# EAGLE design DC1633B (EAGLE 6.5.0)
PROGRAMMABLE HEX VOLTAGE SUPERVISOR WITH EEPROM

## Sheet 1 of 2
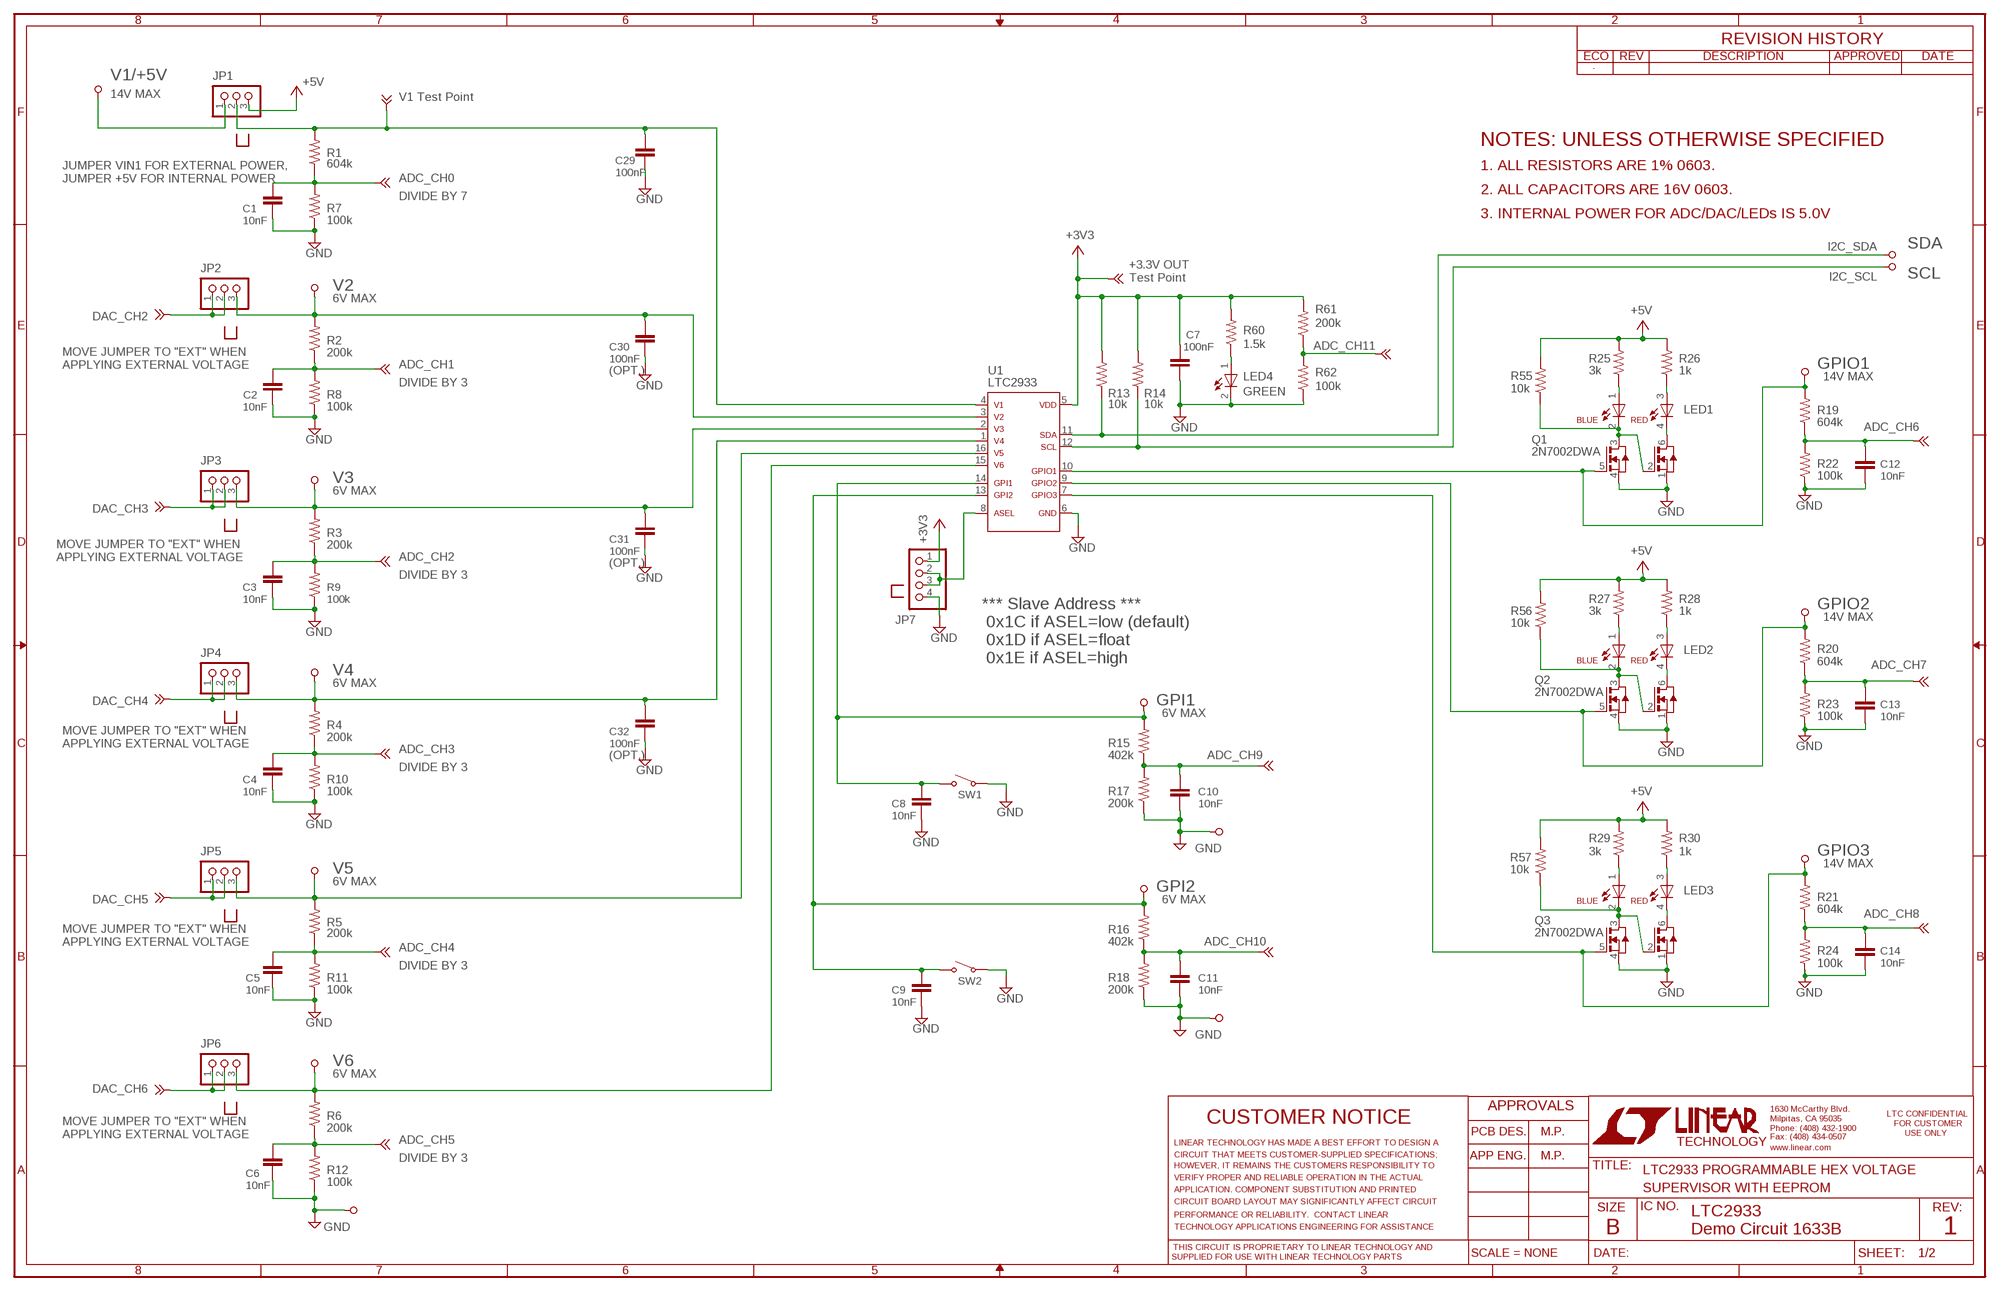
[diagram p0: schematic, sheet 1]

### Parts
C1  10nF  CC0603_BOX  [C0603_BOX]
C2  10nF  CC0603_BOX  [C0603_BOX]
C3  10nF  CC0603_BOX  [C0603_BOX]
C4  10nF  CC0603_BOX  [C0603_BOX]
C5  10nF  CC0603_BOX  [C0603_BOX]
C6  10nF  CC0603_BOX  [C0603_BOX]
C7  100nF  CC0603_BOX  [C0603_BOX]
C8  10nF  CC0603_BOX  [C0603_BOX]
C9  10nF  CC0603_BOX  [C0603_BOX]
C10  10nF  CC0603_BOX  [C0603_BOX]
C11  10nF  CC0603_BOX  [C0603_BOX]
C12  10nF  CC0603_BOX  [C0603_BOX]
C13  10nF  CC0603_BOX  [C0603_BOX]
C14  10nF  CC0603_BOX  [C0603_BOX]
C29  100nF  CC0603_BOX  [C0603_BOX]
C30  100nF  CC0603_BOX  [C0603_BOX]
C31  100nF  CC0603_BOX  [C0603_BOX]
C32  100nF  CC0603_BOX  [C0603_BOX]
JP1  NRPN031PAEN-RC  PINHD-1X3  [1X03]
JP2  NRPN031PAEN-RC  PINHD-1X3  [1X03]
JP3  NRPN031PAEN-RC  PINHD-1X3  [1X03]
JP4  NRPN031PAEN-RC  PINHD-1X3  [1X03]
JP5  NRPN031PAEN-RC  PINHD-1X3  [1X03]
JP6  NRPN031PAEN-RC  PINHD-1X3  [1X03]
JP7  NRPN041PAEN-RC  PINHD-1X4-2MM  [1X04-2MM]
LED1  LED-DUAL-COLOR_1.6X0.8MM  [LED-DUAL_1.6X0.8MM]
LED2  LED-DUAL-COLOR_1.6X0.8MM  [LED-DUAL_1.6X0.8MM]
LED3  LED-DUAL-COLOR_1.6X0.8MM  [LED-DUAL_1.6X0.8MM]
LED4  LED-0603  [CHIPLED_0603]
Q1  2N7002DWA  [SOT-363]
Q2  2N7002DWA  [SOT-363]
Q3  2N7002DWA  [SOT-363]
R1  604k  RR0603_BOX  [R0603_BOX]
R2  200k  RR0603_BOX  [R0603_BOX]
R3  200k  RR0603_BOX  [R0603_BOX]
R4  200k  RR0603_BOX  [R0603_BOX]
R5  200k  RR0603_BOX  [R0603_BOX]
R6  200k  RR0603_BOX  [R0603_BOX]
R7  100k  RR0603_BOX  [R0603_BOX]
R8  100k  RR0603_BOX  [R0603_BOX]
R9  100k  RR0603_BOX  [R0603_BOX]
R10  100k  RR0603_BOX  [R0603_BOX]
R11  100k  RR0603_BOX  [R0603_BOX]
R12  100k  RR0603_BOX  [R0603_BOX]
R13  10k  RR0603_BOX  [R0603_BOX]
R14  10k  RR0603_BOX  [R0603_BOX]
R15  402k  RR0603_BOX  [R0603_BOX]
R16  402k  RR0603_BOX  [R0603_BOX]
R17  200k  RR0603_BOX  [R0603_BOX]
R18  200k  RR0603_BOX  [R0603_BOX]
R19  604k  RR0603_BOX  [R0603_BOX]
R20  604k  RR0603_BOX  [R0603_BOX]
R21  604k  RR0603_BOX  [R0603_BOX]
R22  100k  RR0603_BOX  [R0603_BOX]
R23  100k  RR0603_BOX  [R0603_BOX]
R24  100k  RR0603_BOX  [R0603_BOX]
R25  3k  RR0603_BOX  [R0603_BOX]
R26  1k  RR0603_BOX  [R0603_BOX]
R27  3k  RR0603_BOX  [R0603_BOX]
R28  1k  RR0603_BOX  [R0603_BOX]
R29  3k  RR0603_BOX  [R0603_BOX]
R30  1k  RR0603_BOX  [R0603_BOX]
R55  10k  RR0603_BOX  [R0603_BOX]
R56  10k  RR0603_BOX  [R0603_BOX]
R57  10k  RR0603_BOX  [R0603_BOX]
R60  1.5k  RR0603_BOX  [R0603_BOX]
R61  200k  RR0603_BOX  [R0603_BOX]
R62  100k  RR0603_BOX  [R0603_BOX]
SW1  SWITCH_PTS635  [SWITCH_PTS635]
SW2  SWITCH_PTS635  [SWITCH_PTS635]
TP1  TESTPOINT_BIG  [TP1]
TP2  TESTPOINT_BIG  [TP1]
TP3  TESTPOINT_BIG  [TP1]
TP4  TESTPOINT_BIG  [TP1]
TP5  TESTPOINT_BIG  [TP1]
TP6  TESTPOINT_BIG  [TP1]
TP7  TESTPOINT_BIG  [TP1]
TP8  TESTPOINT_BIG  [TP1]
TP9  TESTPOINT_BIG  [TP1]
TP10  TESTPOINT_BIG  [TP1]
TP11  TESTPOINT_BIG  [TP1]
TP12  TESTPOINT_BIG  [TP1]
TP13  TESTPOINT_BIG  [TP1]
TP14  TESTPOINT_BIG  [TP1]
TP15  TESTPOINT_BIG  [TP1]
TP16  TESTPOINT_BIG  [TP1]
TP20  TESPOINT_SMDVIA  [VIA]
TP21  TESPOINT_SMDVIA  [VIA]
U1  LTC2933  [SSOP16]

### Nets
+3V3: C7.1 JP7.1 R13.2 R14.2 R60.2 R61.2 TP20.1 U1.5
+5V: JP1.3 R25.2 R26.2 R27.2 R28.2 R29.2 R30.2 R55.2 R56.2 R57.2 ; also sheet 2
ADC_CH0: C1.1 R1.1 R7.2 ; also sheet 2
ADC_CH1: C2.1 R2.1 R8.2 ; also sheet 2
ADC_CH2: C3.1 R3.1 R9.2 ; also sheet 2
ADC_CH3: C4.1 R4.1 R10.2 ; also sheet 2
ADC_CH4: C5.1 R5.1 R11.2 ; also sheet 2
ADC_CH5: C6.1 R6.1 R12.2 ; also sheet 2
ADC_CH6: C12.1 R19.1 R22.2 ; also sheet 2
ADC_CH7: C13.1 R20.1 R23.2 ; also sheet 2
ADC_CH8: C14.1 R21.1 R24.2 ; also sheet 2
ADC_CH9: C10.1 R15.1 R17.2 ; also sheet 2
ADC_CH10: C11.1 R16.1 R18.2 ; also sheet 2
ADC_CH11: R61.1 R62.2 ; also sheet 2
DAC_CH2: JP2.1 JP2.2 ; also sheet 2
DAC_CH3: JP3.1 JP3.2 ; also sheet 2
DAC_CH4: JP4.1 JP4.2 ; also sheet 2
DAC_CH5: JP5.1 JP5.2 ; also sheet 2
DAC_CH6: JP6.1 JP6.2 ; also sheet 2
GND: C1.2 C2.2 C3.2 C4.2 C5.2 C6.2 C7.2 C8.2 C9.2 C10.2 C11.2 C12.2 C13.2 C14.2 C29.2 C30.2 C31.2 C32.2 JP7.4 LED4.N(C) Q1.1(S2) Q1.4(S1) Q2.1(S2) Q2.4(S1) Q3.1(S2) Q3.4(S1) R7.1 R8.1 R9.1 R10.1 R11.1 R12.1 R17.1 R18.1 R22.1 R23.1 R24.1 R62.1 SW1.SW2 SW2.SW2 TP14.TP TP15.TP TP16.TP U1.6 ; also sheet 2
I2C_SCL: R14.1 TP13.TP U1.12 ; also sheet 2
I2C_SDA: R13.1 TP12.TP U1.11 ; also sheet 2
N$15: LED4.P(A) R60.1
N$17: JP1.1 TP1.TP
N$20: C29.1 JP1.2 R1.2 TP21.1 U1.4
N$26: JP7.2 JP7.3 U1.8
N$32: Q2.5(G1) R20.2 TP8.TP U1.9
N$34: LED1.4(C4) Q1.6(D2)
N$36: LED2.2(C2) Q2.2(G2) Q2.3(D1) R56.1
N$37: LED3.2(C2) Q3.2(G2) Q3.3(D1) R57.1
N$38: LED1.2(C2) Q1.2(G2) Q1.3(D1) R55.1
N$40: Q3.5(G1) R21.2 TP9.TP U1.7
N$41: Q1.5(G1) R19.2 TP7.TP U1.10
N$44: LED3.4(C4) Q3.6(D2)
N$45: LED3.1(A1) R29.1
N$47: LED3.3(A3) R30.1
N$49: LED2.4(C4) Q2.6(D2)
N$50: LED2.1(A1) R27.1
N$51: LED2.3(A3) R28.1
N$54: LED1.1(A1) R25.1
N$55: LED1.3(A3) R26.1
N$77: C8.1 R15.2 SW1.SW1 TP10.TP U1.14
N$78: C9.1 R16.2 SW2.SW1 TP11.TP U1.13
VIN2: C30.1 JP2.3 R2.2 TP2.TP U1.3
VIN3: C31.1 JP3.3 R3.2 TP3.TP U1.2
VIN4: C32.1 JP4.3 R4.2 TP4.TP U1.1
VIN5: JP5.3 R5.2 TP5.TP U1.16
VIN6: JP6.3 R6.2 TP6.TP U1.15

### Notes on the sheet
- V1/+5V
- 14V MAX | V1 Test Point
- NOTES: UNLESS OTHERWISE SPECIFIED
- 1. ALL RESISTORS ARE 1% 0603.
- JUMPER VIN1 FOR EXTERNAL POWER,
  JUMPER +5V FOR INTERNAL POWER
- 2. ALL CAPACITORS ARE 16V 0603.
- DIVIDE BY 7
- 3. INTERNAL POWER FOR ADC/DAC/LEDs IS 5.0V
- SDA
- SCL
- +3.3V OUT
  Test Point
- V2
- 6V MAX
- MOVE JUMPER TO "EXT" WHEN
  APPLYING EXTERNAL VOLTAGE
- GPIO1
- (OPT.)
- 14V MAX
- DIVIDE BY 3
- GREEN
- V3
- 6V MAX
- MOVE JUMPER TO "EXT" WHEN
  APPLYING EXTERNAL VOLTAGE
- (OPT.)
- DIVIDE BY 3
- GPIO2
- 14V MAX
- *** Slave Address ***
   0x1C if ASEL=low (default)
   0x1D if ASEL=float
   0x1E if ASEL=high
- V4
- 6V MAX
- GPI1
- 6V MAX
- MOVE JUMPER TO "EXT" WHEN
  APPLYING EXTERNAL VOLTAGE
- (OPT.)
- DIVIDE BY 3
- GPIO3
- 14V MAX
- V5
- 6V MAX
- GPI2
- 6V MAX
- MOVE JUMPER TO "EXT" WHEN
  APPLYING EXTERNAL VOLTAGE
- DIVIDE BY 3
- V6
- 6V MAX
- M.P.
- MOVE JUMPER TO "EXT" WHEN
  APPLYING EXTERNAL VOLTAGE
- DIVIDE BY 3 | M.P.
- LTC2933 PROGRAMMABLE HEX VOLTAGE
- SUPERVISOR WITH EEPROM
- LTC2933
- Demo Circuit 1633B | 1

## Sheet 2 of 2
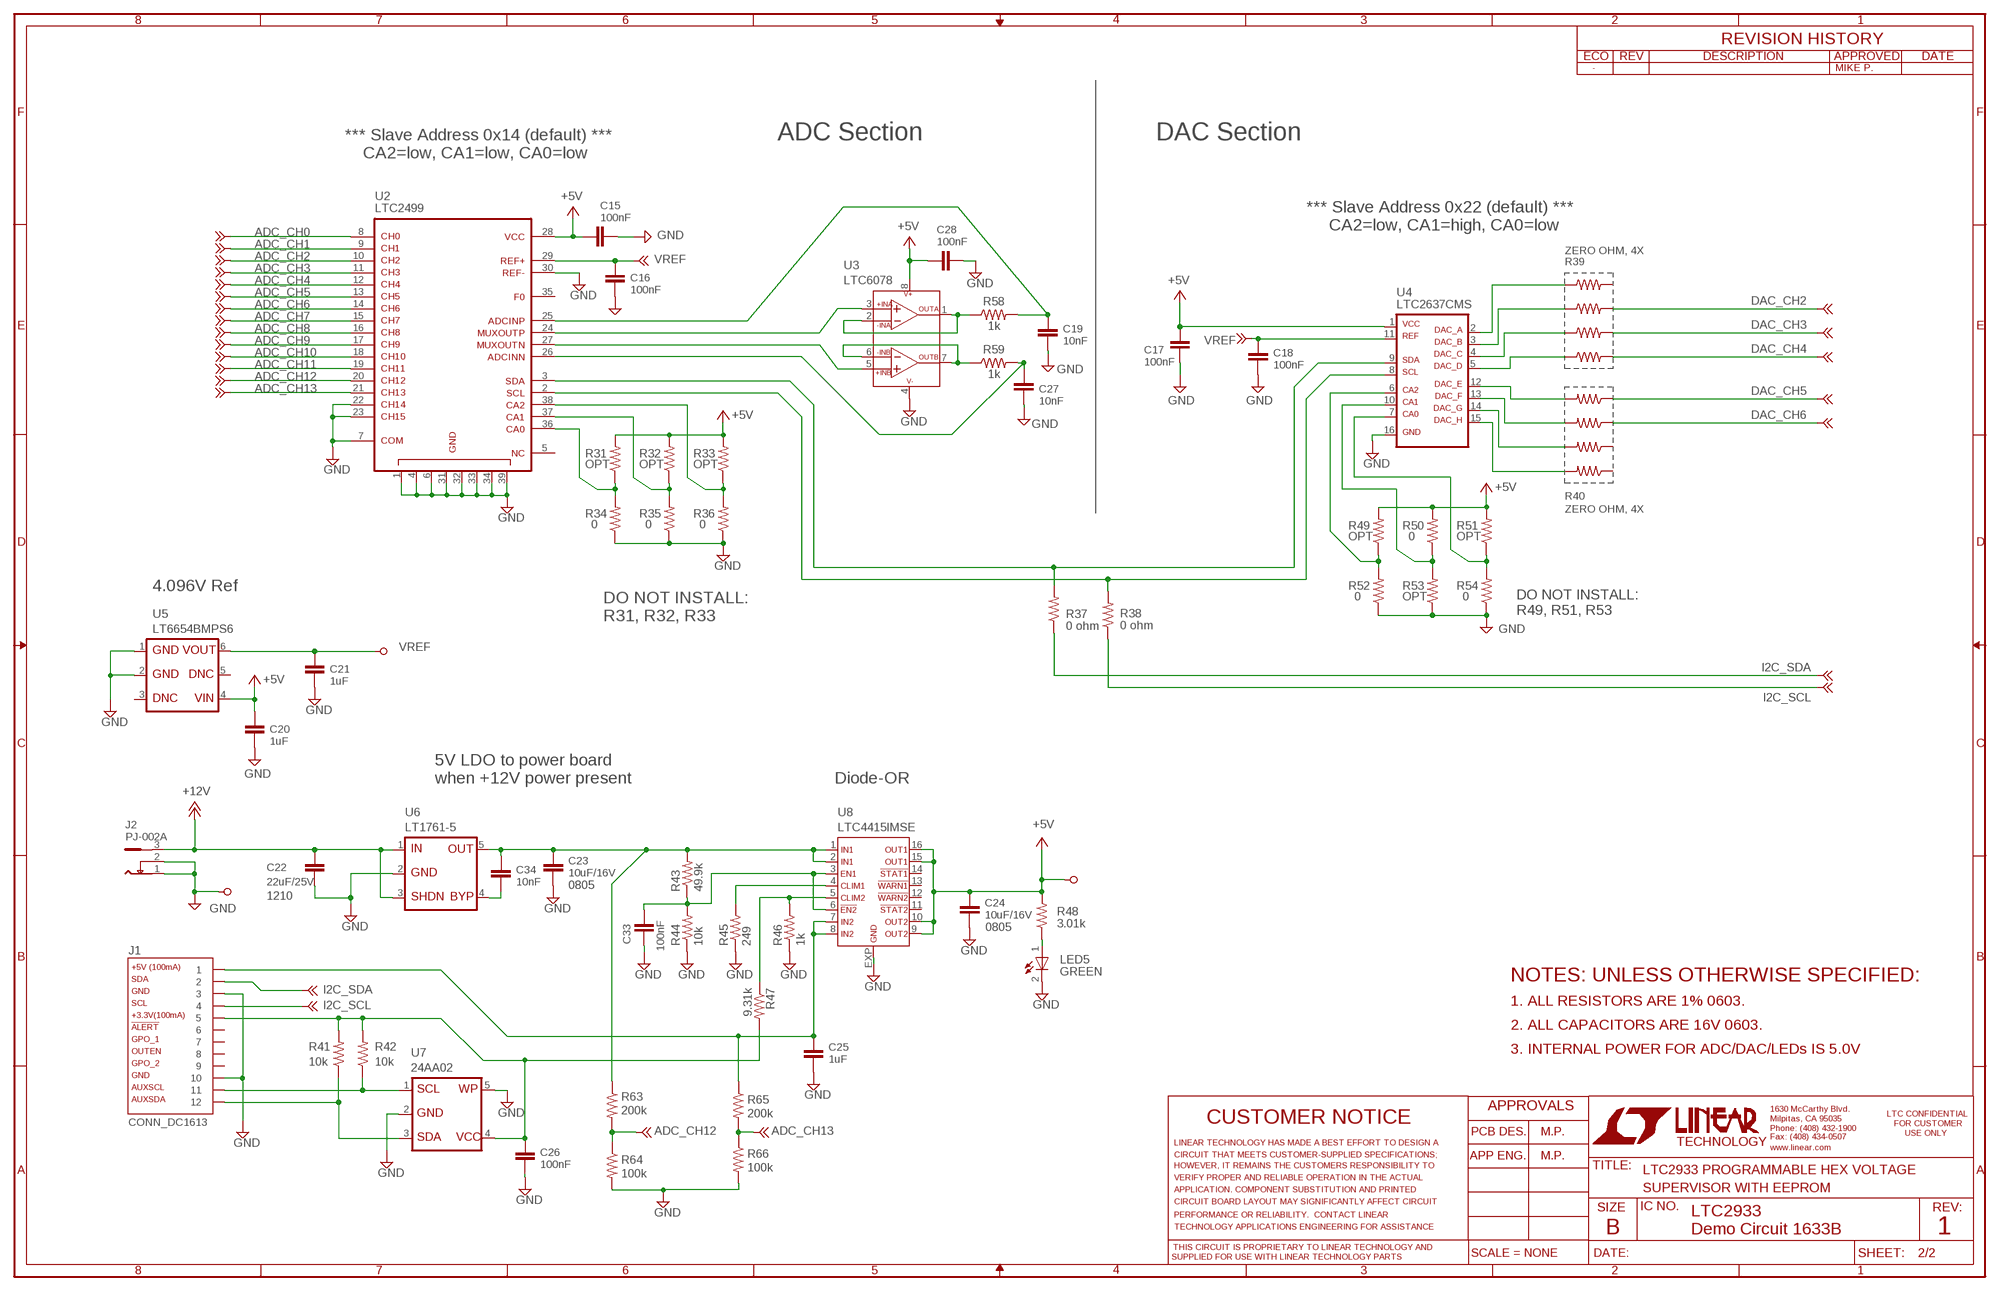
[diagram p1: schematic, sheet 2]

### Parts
C15  100nF  CC0603_BOX  [C0603_BOX]
C16  100nF  CC0603_BOX  [C0603_BOX]
C17  100nF  CC0603_BOX  [C0603_BOX]
C18  100nF  CC0603_BOX  [C0603_BOX]
C19  10nF  CC0603_BOX  [C0603_BOX]
C20  1uF  CC0603_BOX  [C0603_BOX]
C21  1uF  CC0603_BOX  [C0603_BOX]
C22  22uF/25V  CC1210_BOX  [C1210_BOX]
C23  10uF/16V  CC0805_BOX  [C0805_BOX]
C24  10uF/16V  CC0805_BOX  [C0805_BOX]
C25  1uF  CC0603_BOX  [C0603_BOX]
C26  100nF  CC0603_BOX  [C0603_BOX]
C27  10nF  CC0603_BOX  [C0603_BOX]
C28  100nF  CC0603_BOX  [C0603_BOX]
C33  100nF  CC0603_BOX  [C0603_BOX]
C34  10nF  CC0603_BOX  [C0603_BOX]
J1  CONN_DC1613  [CONN_DC1613]
J2  PJ-002A  [PJ-002A]
LED5  LED-0603  [CHIPLED_0603]
R31  OPT  RR0603_BOX  [R0603_BOX]
R32  OPT  RR0603_BOX  [R0603_BOX]
R33  OPT  RR0603_BOX  [R0603_BOX]
R34  0  RR0603_BOX  [R0603_BOX]
R35  0  RR0603_BOX  [R0603_BOX]
R36  0  RR0603_BOX  [R0603_BOX]
R37  0 ohm  RR0603_BOX  [R0603_BOX]
R38  0 ohm  RR0603_BOX  [R0603_BOX]
R39  R_ARRAY_4X_CRA06S  [R_VISHAY_CRA06S]
R40  R_ARRAY_4X_CRA06S  [R_VISHAY_CRA06S]
R41  10k  RR0603_BOX  [R0603_BOX]
R42  10k  RR0603_BOX  [R0603_BOX]
R43  49.9k  RR0603_BOX  [R0603_BOX]
R44  10k  RR0603_BOX  [R0603_BOX]
R45  249  RR0603_BOX  [R0603_BOX]
R46  1k  RR0603_BOX  [R0603_BOX]
R47  9.31k  RR0603_BOX  [R0603_BOX]
R48  3.01k  RR0603_BOX  [R0603_BOX]
R49  OPT  RR0603_BOX  [R0603_BOX]
R50  0  RR0603_BOX  [R0603_BOX]
R51  OPT  RR0603_BOX  [R0603_BOX]
R52  0  RR0603_BOX  [R0603_BOX]
R53  OPT  RR0603_BOX  [R0603_BOX]
R54  0  RR0603_BOX  [R0603_BOX]
R58  1k  RR0603_BOX  [R0603_BOX]
R59  1k  RR0603_BOX  [R0603_BOX]
R63  200k  RR0603_BOX  [R0603_BOX]
R64  100k  RR0603_BOX  [R0603_BOX]
R65  200k  RR0603_BOX  [R0603_BOX]
R66  100k  RR0603_BOX  [R0603_BOX]
TP17  TESTPOINT_BIG  [TP1]
TP18  TESTPOINT_BIG  [TP1]
TP19  TURRET_SMALL_2308TP  [TURRET_SMALL_2308]
TP24  TESPOINT_SMDVIA  [VIA]
TP25  TESPOINT_SMDVIA  [VIA]
TP26  TESPOINT_SMDVIA  [VIA]
TP27  TESPOINT_SMDVIA  [VIA]
TP28  TESPOINT_SMDVIA  [VIA]
TP29  TESPOINT_SMDVIA  [VIA]
TP33  TESPOINT_SMDVIA  [VIA]
TP34  TESPOINT_SMDVIA  [VIA]
U2  LTC2499  [QFN38_5X7]
U3  LTC6078  [MSOP8]
U4  LTC2637CMS  [MSOP16]
U5  LT6654BMPS6  [SOT-23-6]
U6  LT1761-5  [SOT-23-5]
U7  24AA02  [SOT-23-5]
U8  LTC4415IMSE  [MSOP16_EXP]

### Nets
+5V: C15.1 C17.1 C20.1 C24.1 C28.1 R31.2 R32.2 R33.2 R48.2 R49.2 R50.2 R51.2 TP18.TP U2.28 U3.8 U4.1 U5.4 U8.9 U8.10 U8.15 U8.16 ; also sheet 1
+12V: C22.1 J2.3 U6.1 U6.3
ADC_CH0: TP24.1 U2.8 ; also sheet 1
ADC_CH1: TP25.1 U2.9 ; also sheet 1
ADC_CH2: TP26.1 U2.10 ; also sheet 1
ADC_CH3: TP27.1 U2.11 ; also sheet 1
ADC_CH4: TP28.1 U2.12 ; also sheet 1
ADC_CH5: TP29.1 U2.13 ; also sheet 1
ADC_CH6: U2.14 ; also sheet 1
ADC_CH7: U2.15 ; also sheet 1
ADC_CH8: U2.16 ; also sheet 1
ADC_CH9: TP33.1 U2.17 ; also sheet 1
ADC_CH10: TP34.1 U2.18 ; also sheet 1
ADC_CH11: U2.19 ; also sheet 1
ADC_CH12: R63.2 R64.1 U2.20
ADC_CH13: R65.2 R66.1 U2.21
DAC_CH2: R39.R2_2 ; also sheet 1
DAC_CH3: R39.R3_2 ; also sheet 1
DAC_CH4: R39.R4_2 ; also sheet 1
DAC_CH5: R40.R4_1 ; also sheet 1
DAC_CH6: R40.R3_1 ; also sheet 1
GND: C15.2 C16.2 C17.2 C18.2 C19.2 C20.2 C21.2 C22.2 C23.2 C24.2 C25.2 C26.2 C27.2 C28.2 C33.2 J1.3 J1.10 J2.1 J2.2 LED5.N(C) R34.1 R35.1 R36.1 R44.1 R45.1 R46.1 R52.1 R53.1 R54.1 R64.2 R66.2 TP17.TP U2.1(GND1) U2.4(GND4) U2.6(GND6) U2.7 U2.22 U2.23 U2.30 U2.31(GND31) U2.32(GND32) U2.33(GND33) U2.34(GND34) U2.39(GND39) U3.4 U4.16 U5.1 U5.2 U6.2 U7.2 U7.5 U8.EXP ; also sheet 1
I2C_SCL: J1.4 R38.1 ; also sheet 1
I2C_SDA: J1.2 R37.1 ; also sheet 1
N$1: R40.R4_2 U4.12
N$2: R50.1 R53.2 U4.10
N$3: R40.R3_2 U4.13
N$4: R51.1 R54.2 U4.7
N$5: R40.R2_2 U4.14
N$6: R49.1 R52.2 U4.6
N$7: R40.R1_2 U4.15
N$9: R39.R4_1 U4.5
N$10: LED5.P(A) R48.1
N$11: R39.R3_1 U4.4
N$12: C23.1 C34.1 R43.2 R63.1 U6.5 U8.1 U8.2
N$13: R39.R2_1 U4.3
N$14: C33.1 R43.1 R44.2 U8.3 U8.6
N$16: R58.1 U3.1 U3.2
N$18: R39.R1_1 U4.2
N$19: R38.2 U2.2 U4.8
N$21: R45.2 U8.4
N$22: R46.2 R47.1 U8.5
N$23: C34.2 U6.4
N$24: J1.11 R42.1 U7.1
N$25: J1.12 R41.1 U7.3
N$27: R32.1 R35.2 U2.37
N$28: R31.1 R34.2 U2.36
N$29: R37.2 U2.3 U4.9
N$30: R33.1 R36.2 U2.38
N$31: U2.24 U3.3
N$33: U2.27 U3.5
N$39: R59.1 U3.6 U3.7
N$43: C26.1 J1.5 R41.2 R42.2 R47.2 U7.4
N$46: C27.1 R59.2 U2.26
N$48: C19.1 R58.2 U2.25
USB_5V: C25.1 J1.1 R65.1 U8.7 U8.8
VREF: C16.1 C18.1 C21.1 TP19.TP1 U2.29 U4.11 U5.6
Unconnected: J1.6 J1.7 J1.8 J1.9 R39.R1_2 R40.R1_1 R40.R2_1 U2.5 U2.35 U5.3 U5.5 U8.11 U8.12 U8.13 U8.14

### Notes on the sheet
- MIKE P.
- ADC Section | DAC Section
- *** Slave Address 0x14 (default) ***
      CA2=low, CA1=low, CA0=low
- *** Slave Address 0x22 (default) ***
       CA2=low, CA1=high, CA0=low
- ZERO OHM, 4X
- ZERO OHM, 4X
- 4.096V Ref
- DO NOT INSTALL:
  R49, R51, R53
- DO NOT INSTALL:
  R31, R32, R33
- 5V LDO to power board
  when +12V power present
- Diode-OR
- 0805
- 1210
- 0805
- GREEN
- NOTES: UNLESS OTHERWISE SPECIFIED:
- 1. ALL RESISTORS ARE 1% 0603.
- 2. ALL CAPACITORS ARE 16V 0603.
- 3. INTERNAL POWER FOR ADC/DAC/LEDs IS 5.0V
- M.P.
- M.P.
- LTC2933 PROGRAMMABLE HEX VOLTAGE
- SUPERVISOR WITH EEPROM
- LTC2933
- Demo Circuit 1633B | 1

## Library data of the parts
C1-C34 = kalin:C: CAPACITOR, European symbol
J1 = kalin:CONN_DC1613: Connector for LT DC1613 USB Dongle
J2 = kalin:PJ-002A: Power Jack from CUI Inc. PJ-002A
JP1-JP6 = pinhead:PINHD-1X3: PIN HEADER
JP7 = pinhead:PINHD-1X4-2MM: PIN HEADER
LED1-LED3 = kalin:LED-DUAL-COLOR_1.6X0.8MM
LED4 LED5 = kalin:LED-0603: SMD LED in R0603
Q1-Q3 = kalin:2N7002DWA
R1-R38 R41-R66 = kalin:R: RESISTOR, American symbol
R39 R40 = kalin:R_ARRAY_4X_CRA06S: Thick Film Resistor Array
SW1 SW2 = kalin:SWITCH_PTS635: PTS635SL25 Surface Mount Tactile Switch
TP1-TP18 = kalin:TESTPOINT_BIG: Large Test Point
TP19 = kalin:TURRET_SMALL_2308: Small Test Turret Mill-Max 2308
TP20 TP21 TP24-TP29 TP33 TP34 = kalin:TESPOINT_SMD: SMALL SMD Test Point
U1 = kalin:LTC2933: Programmable Hex Voltage Supervisor with EEPROM
U2 = kalin:LTC2499: 24-BIT 16-CHANNEL DELTA SIGMA ADC WITH I2C INTERFACE
U3 = kalin:LTC6078: Micropower Precision Rail-to-Rail Dual Op-Amp
U4 = kalin:LTC2637CMS
U5 = kalin:LT6654: SOT-23 Precision Wide Supply High Output Drive Low Noise Reference
U6 = kalin:LT1761-5: 100mA, Low Noise, LDO Micropower Regulators in TSOT-23
U7 = kalin:24AA02: 2Kbit I2C Serial EEPROM
U8 = kalin:LTC4415: Dual 4A Ideal Diodes with Adjustable Current Limit

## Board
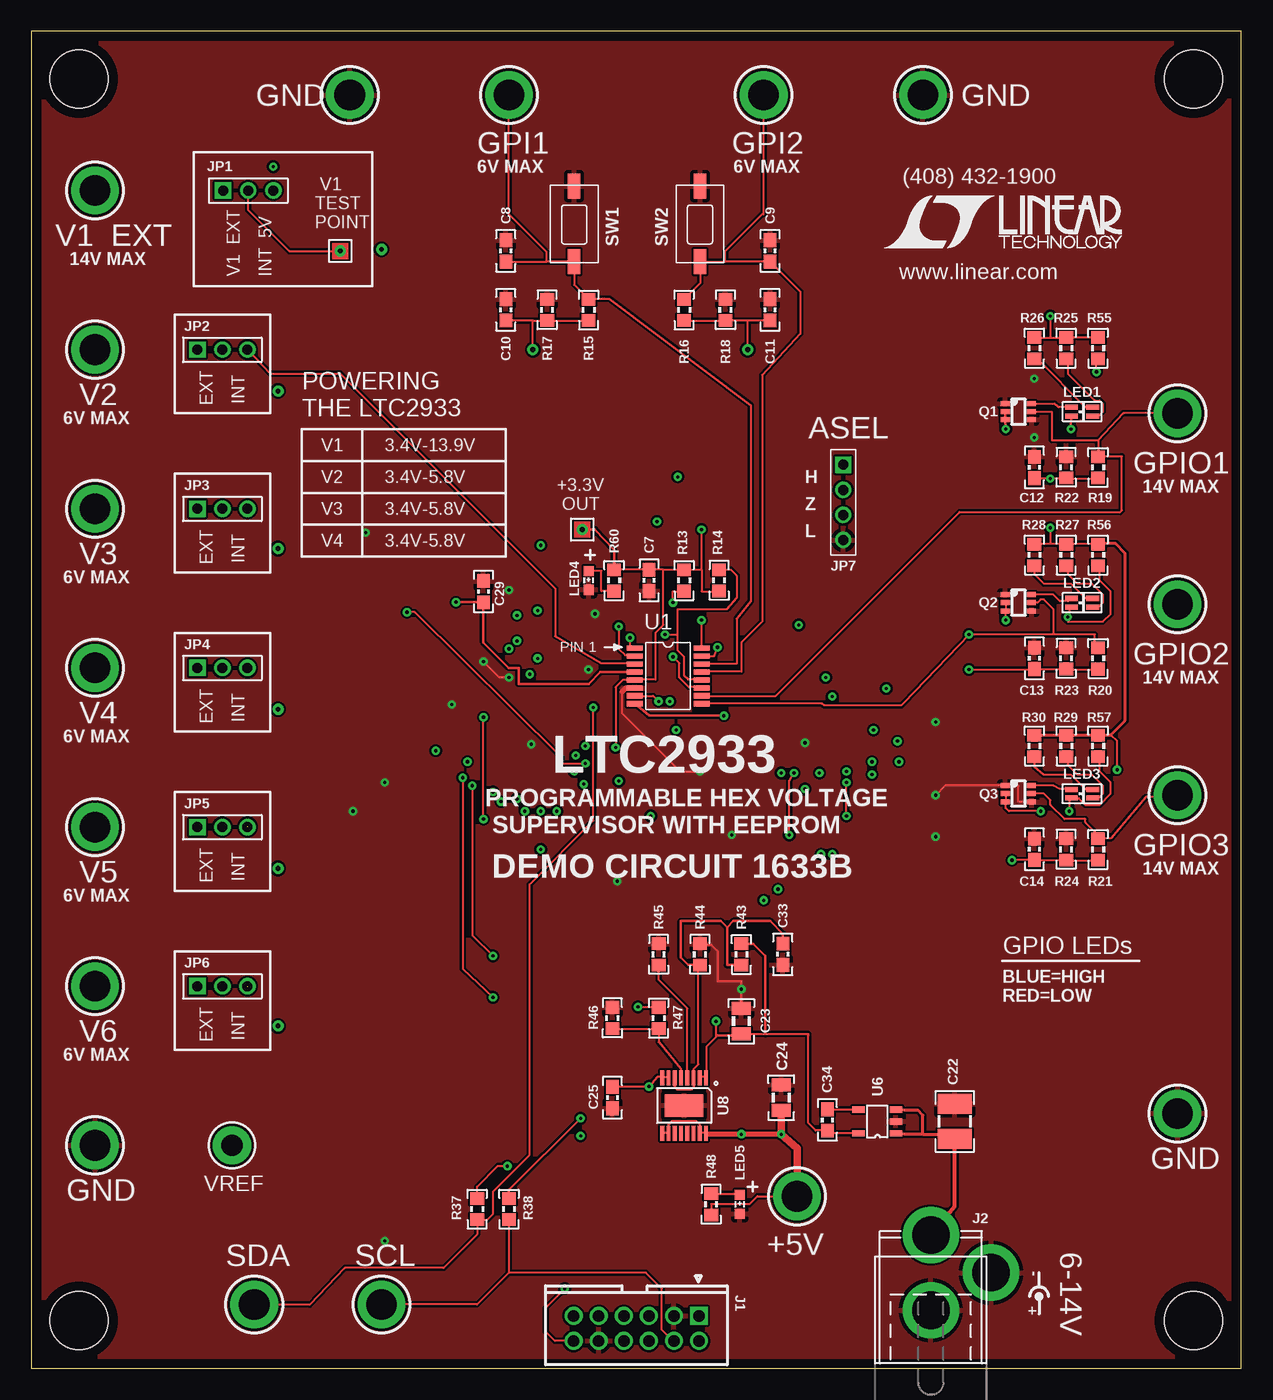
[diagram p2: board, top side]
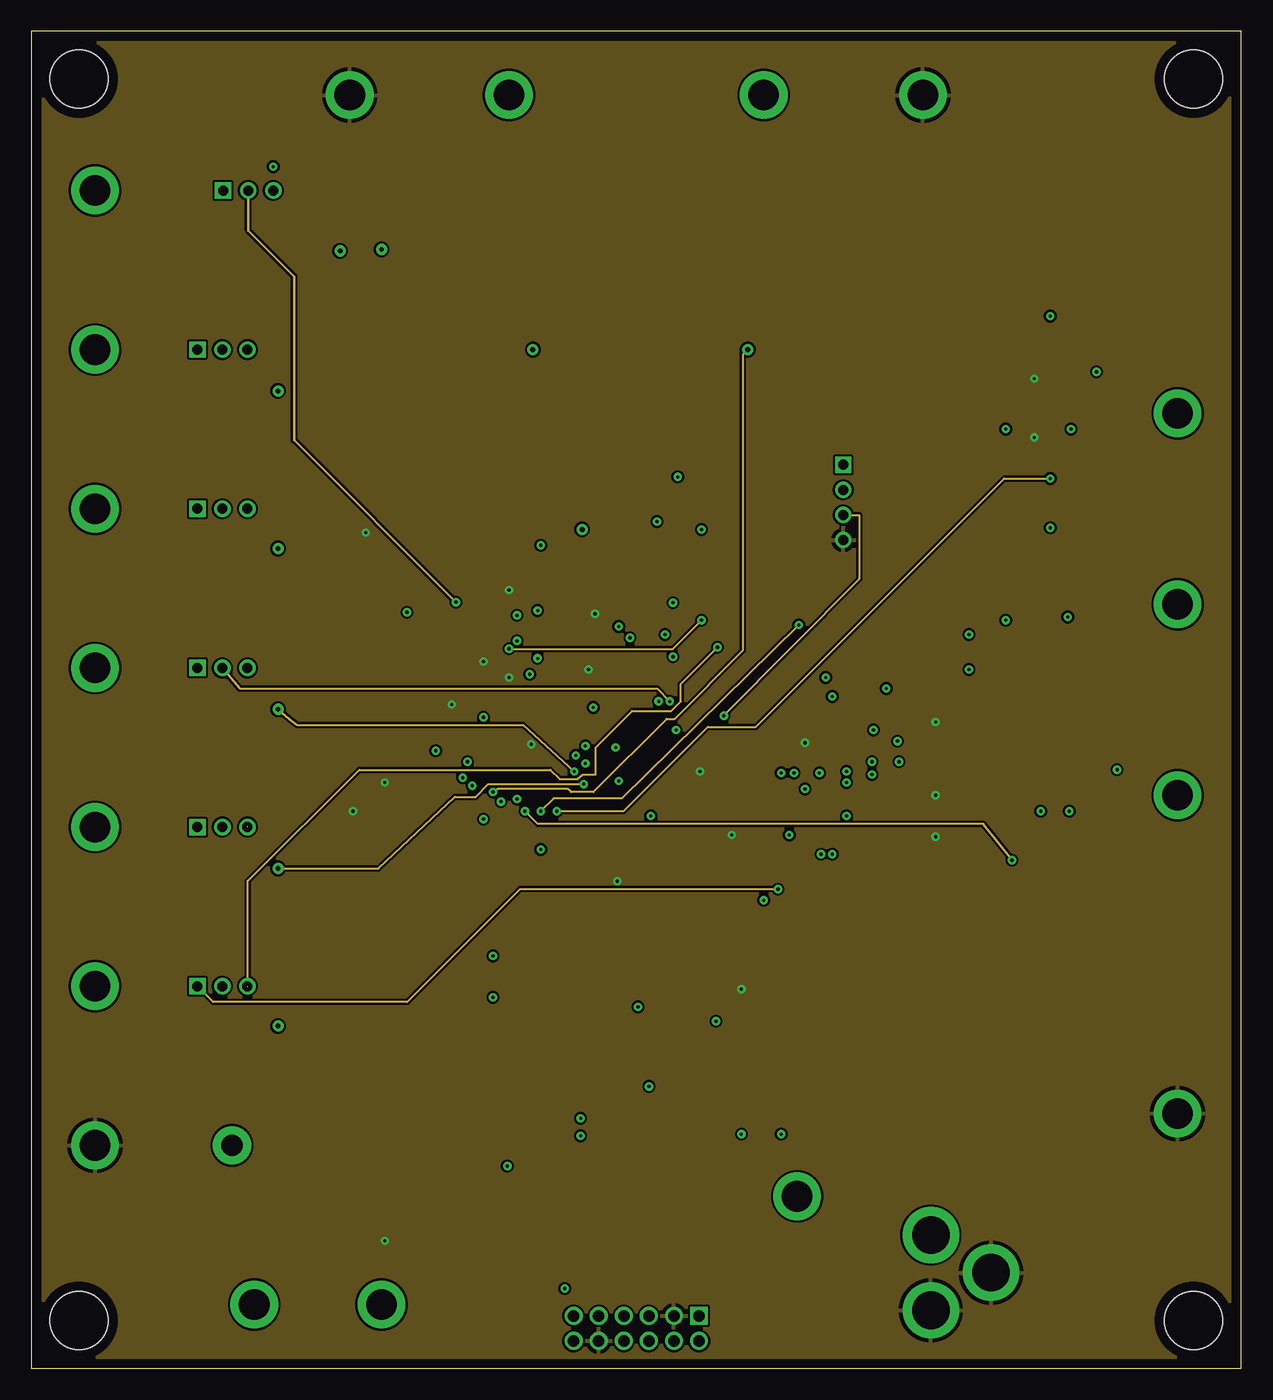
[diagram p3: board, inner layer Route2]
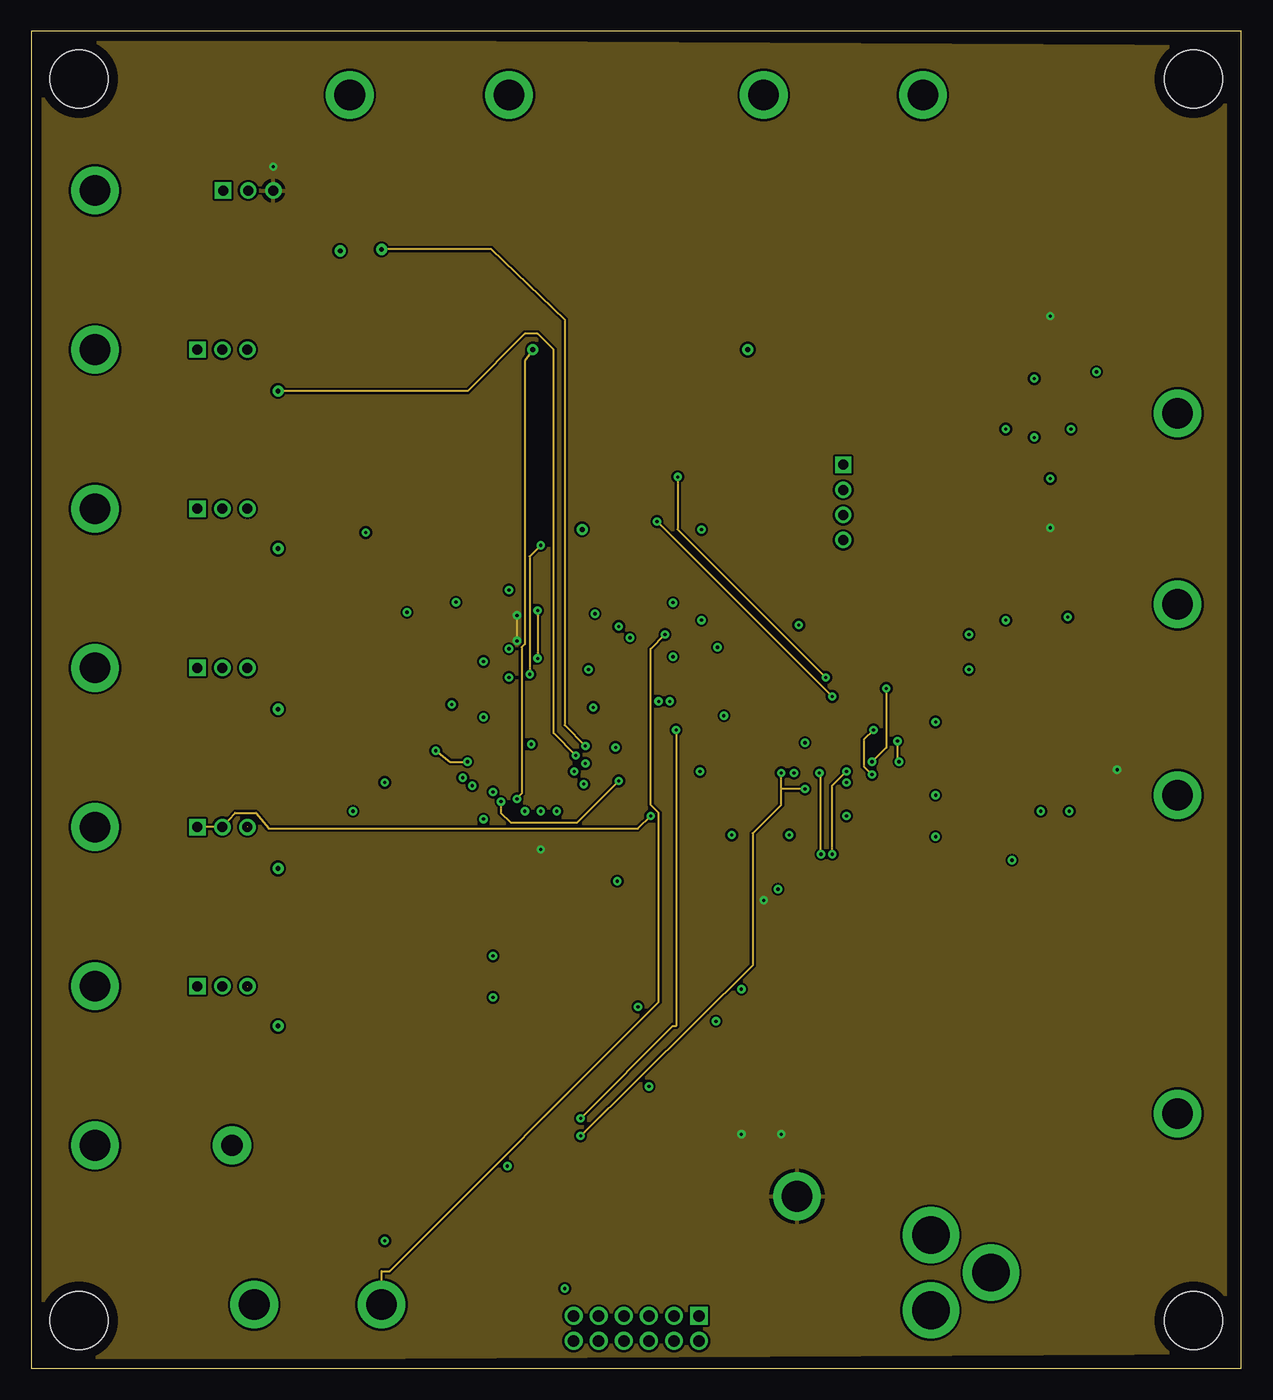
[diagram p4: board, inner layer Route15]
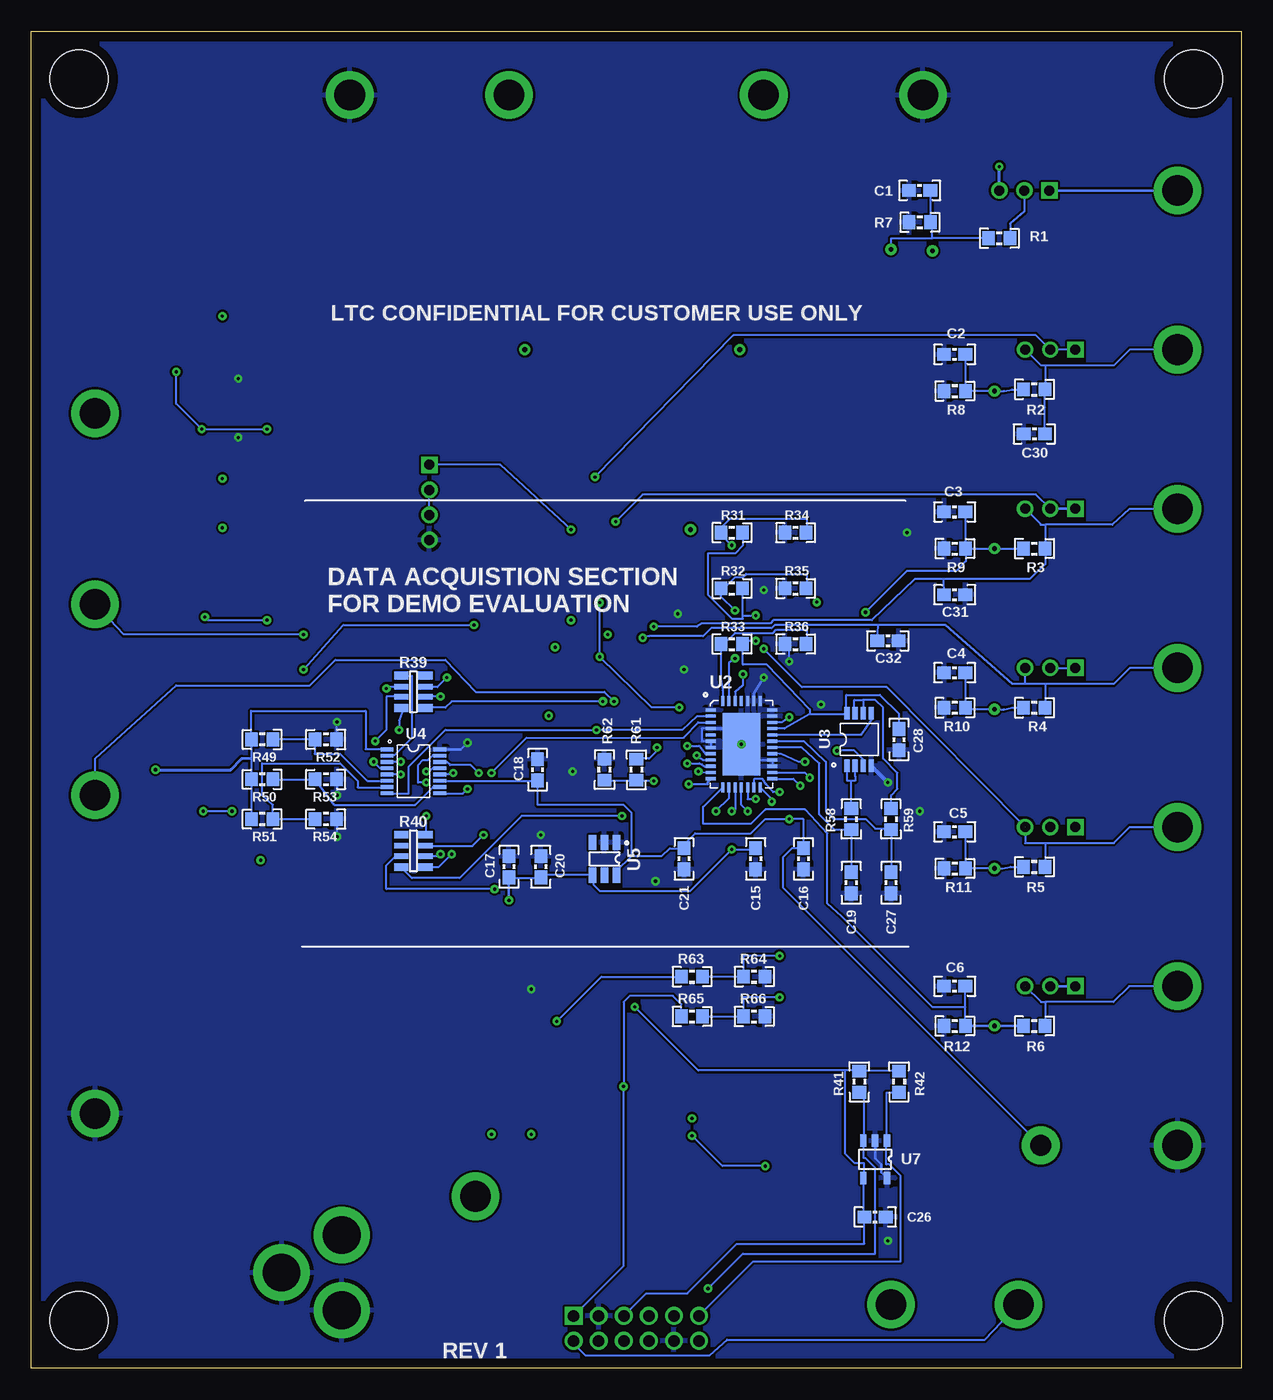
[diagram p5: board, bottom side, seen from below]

Size 96.52 x 106.68 mm. Coordinates in mm from the lower left corner, seen from the top.
Outline: 0,0 96.52,0 96.52,106.68 0,106.68 0,0
Copper layers (1*2+15*16): Top 0.06858125mm / dielectric 9mil / Route2 0.034290625mm / dielectric 0.911859375mm / Route15 0.034290625mm / dielectric 9mil / Bottom 0.06858125mm
Design rules "default *": minimum track width 7mil, minimum drill 10mil, track to track 7mil, track to pad 6mil, pad to pad 7mil, via to via 7mil, smd to smd 4mil, copper to edge 30mil, drill to drill 15mil, minimum pad ring 10mil, minimum via ring 8mil, stop-mask expansion 4mil, vias tented up to drill 10mil, thermal gap 12mil
Holes 4.65 mm at 3.81,3.81 92.71,3.81 92.71,102.87 3.81,102.87

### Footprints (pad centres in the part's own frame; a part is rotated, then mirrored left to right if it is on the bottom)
C0603_BOX = smd 1.1 x 1: 1 -0.85,0; 2 0.85,0
C1210_BOX = smd 1.6 x 2.7: 1 -1.4,0; 2 1.4,0
C0805_BOX = smd 1.016 x 1.524: 1 -1.016,0; 2 1.016,0
CONN_DC1613 = drill 0.914 square: 1 -5,-1 | drill 0.914: 2 -5,1; 3 -3,-1; 4 -3,1; 5 -1,-1; 6 -1,1; 7 1,-1; 8 1,1; 9 3,-1; 10 3,1; 11 5,-1; 12 5,1
PJ-002A = drill 3 pad 4.5: 1 -3,0; 2 0,-4.8; 3 3,0
1X03 = drill 0.8 square: 1 -2,0 | drill 0.8: 2 0,0; 3 2,0
1X04-2MM = drill 0.8 square: 1 -3,0 | drill 0.8: 2 -1,0; 3 1,0; 4 3,0
LED-DUAL_1.6X0.8MM = smd 1 x 0.4: 1 0.85,-0.35; 2 -0.85,-0.35; 3 0.85,0.35; 4 -0.85,0.35
CHIPLED_0603 = smd 0.8 x 0.8: N 0,0.75; P 0,-0.75
SOT-363 = smd 0.7 x 0.4: 1 -1.05,0.65; 2 -1.05,0; 3 -1.05,-0.65; 4 1.05,-0.65; 5 1.05,0; 6 1.05,0.65
R0603_BOX = smd 1 x 1.1: 1 -0.85,0; 2 0.85,0
R_VISHAY_CRA06S = smd 1.15 x 0.63: R1_1 -0.975,1.295; R1_2 0.975,1.295; R4_1 -0.975,-1.295; R4_2 0.975,-1.295 | smd 1.15 x 0.44: R2_1 -0.975,0.4; R2_2 0.975,0.4; R3_1 -0.975,-0.4; R3_2 0.975,-0.4
SWITCH_PTS635 = smd 2 x 1: SW1 -3,0; SW2 3,0
TP1 = drill 2.438 pad 3.81: TP 0,0
TURRET_SMALL_2308 = drill 1.702 pad 3.048: TP1 0,0
VIA = drill 0.381: 1 0,0
SSOP16 = smd 1.27 x 0.406: 1 -2.667,2.223; 2 -2.667,1.587; 3 -2.667,0.953; 4 -2.667,0.318; 5 -2.667,-0.318; 6 -2.667,-0.953; 7 -2.667,-1.587; 8 -2.667,-2.223; 9 2.667,-2.223; 10 2.667,-1.587; 11 2.667,-0.953; 12 2.667,-0.318; 13 2.667,0.318; 14 2.667,0.953; 15 2.667,1.587; 16 2.667,2.223
QFN38_5X7 = smd 0.8 x 0.25: 1 -2.45,2.75; 2 -2.45,2.25; 3 -2.45,1.75; 4 -2.45,1.25; 5 -2.45,0.75; 6 -2.45,0.25; 7 -2.45,-0.25; 8 -2.45,-0.75; 9 -2.45,-1.25; 10 -2.45,-1.75; 11 -2.45,-2.25; 12 -2.45,-2.75; 20 2.45,-2.75; 21 2.45,-2.25; 22 2.45,-1.75; 23 2.45,-1.25; 24 2.45,-0.75; 25 2.45,-0.25; 26 2.45,0.25; 27 2.45,0.75; 28 2.45,1.25; 29 2.45,1.75; 30 2.45,2.25; 31 2.45,2.75 | smd 0.25 x 0.8: 13 -1.5,-3.45; 14 -1,-3.45; 15 -0.5,-3.45; 16 0,-3.45; 17 0.5,-3.45; 18 1,-3.45; 19 1.5,-3.45; 32 1.5,3.45; 33 1,3.45; 34 0.5,3.45; 35 0,3.45; 36 -0.5,3.45; 37 -1,3.45; 38 -1.5,3.45 | smd 3 x 5: 39 0,0
MSOP8 = smd 0.42 x 1: 1 -0.98,-2.1; 2 -0.33,-2.1; 3 0.32,-2.1; 4 0.97,-2.1; 5 0.97,2.1; 6 0.32,2.1; 7 -0.33,2.1; 8 -0.98,2.1
MSOP16 = smd 0.3 x 1: 1 -1.75,-2.1; 2 -1.25,-2.1; 3 -0.75,-2.1; 4 -0.25,-2.1; 5 0.25,-2.1; 6 0.75,-2.1; 7 1.25,-2.1; 8 1.75,-2.1; 9 1.75,2.1; 10 1.25,2.1; 11 0.75,2.1; 12 0.25,2.1; 13 -0.25,2.1; 14 -0.75,2.1; 15 -1.25,2.1; 16 -1.75,2.1
SOT-23-6 = smd 1.2 x 0.6: 1 -1.3,0.95; 2 -1.3,0; 3 -1.3,-0.95; 4 1.3,-0.95; 5 1.3,0; 6 1.3,0.95
SOT-23-5 = smd 1 x 0.5: 1 -1.649,0.95; 2 -1.649,0; 3 -1.649,-0.95; 4 1.333,-0.95; 5 1.333,0.95
MSOP16_EXP = smd 1.2 x 0.3: 1 -2.213,1.75; 2 -2.213,1.25; 3 -2.213,0.75; 4 -2.213,0.25; 5 -2.213,-0.25; 6 -2.213,-0.75; 7 -2.213,-1.25; 8 -2.213,-1.75; 9 2.213,-1.75; 10 2.213,-1.25; 11 2.213,-0.75; 12 2.213,-0.25; 13 2.213,0.25; 14 2.213,0.75; 15 2.213,1.25; 16 2.213,1.75 | smd 1.778 x 3.048: EXP 0,0

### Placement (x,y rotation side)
C1  25.65,93.98 180 bottom
C2  22.86,80.9 180 bottom
C3  22.86,68.33 180 bottom
C4  22.86,55.5 180 bottom
C5  22.86,42.8 180 bottom
C6  22.86,30.48 180 bottom
C7  49.28,62.87 270 top
C8  37.85,89.15 90 top
C9  58.93,89.15 90 top
C10  37.85,84.45 90 top
C11  58.93,84.45 90 top
C12  80.01,71.88 90 top
C13  80.01,56.64 90 top
C14  80.01,41.4 90 top
C15  38.73,40.64 270 bottom
C16  34.92,40.64 270 bottom
C17  58.42,40.01 90 bottom
C18  56.13,47.75 90 bottom
C19  31.11,38.73 270 bottom
C20  55.88,40.01 90 bottom
C21  44.45,40.64 270 bottom
C22  73.66,19.68 90 top
C23  56.64,27.69 90 top
C24  59.82,21.59 90 top
C25  46.35,21.59 270 top
C26  29.21,12.06 0 bottom
C27  27.94,38.73 270 bottom
C28  27.3,50.16 270 bottom
C29  36.07,61.98 90 top
C30  16.51,74.55 180 bottom
C31  22.86,61.72 0 bottom
C32  28.19,58.04 0 bottom
C33  59.94,33.02 270 top
C34  63.5,19.81 90 top
J1  48.26,3.17 180 top
J2  71.75,7.62 90 top
JP1  17.3,93.98 0 top
JP2  15.24,81.28 0 top
JP3  15.24,68.58 0 top
JP4  15.24,55.88 0 top
JP5  15.24,43.18 0 top
JP6  15.24,30.48 0 top
JP7  64.77,69.09 270 top
LED1  83.82,76.33 0 top
LED2  83.82,61.09 0 top
LED3  83.82,45.85 0 top
LED4  44.45,62.87 180 top
LED5  56.52,13.08 180 top
Q1  78.74,76.33 0 top
Q2  78.74,61.09 0 top
Q3  78.74,45.85 0 top
R1  19.3,90.17 0 bottom
R2  16.51,78.11 0 bottom
R3  16.51,65.41 0 bottom
R4  16.51,52.7 0 bottom
R5  16.51,40.01 0 bottom
R6  16.51,27.3 0 bottom
R7  25.65,91.44 0 bottom
R8  22.86,77.98 0 bottom
R9  22.86,65.41 0 bottom
R10  22.86,52.7 0 bottom
R11  22.86,39.88 0 bottom
R12  22.86,27.3 0 bottom
R13  52.07,62.87 90 top
R14  54.86,62.87 270 top
R15  44.45,84.45 90 top
R16  52.07,84.45 90 top
R17  41.15,84.45 270 top
R18  55.37,84.45 270 top
R19  85.09,71.88 90 top
R20  85.09,56.64 90 top
R21  85.09,41.4 90 top
R22  82.55,71.88 270 top
R23  82.55,56.64 270 top
R24  82.55,41.4 270 top
R25  82.55,81.41 90 top
R26  80.01,81.41 90 top
R27  82.55,64.9 90 top
R28  80.01,64.9 90 top
R29  82.55,49.66 90 top
R30  80.01,49.66 90 top
R31  40.64,66.67 0 bottom
R32  40.64,62.23 0 bottom
R33  40.64,57.78 0 bottom
R34  35.56,66.67 0 bottom
R35  35.56,62.23 0 bottom
R36  35.56,57.78 0 bottom
R37  35.56,12.7 90 top
R38  38.1,12.7 90 top
R39  66.04,53.98 0 bottom
R40  66.04,41.27 0 bottom
R41  30.48,22.86 90 bottom
R42  27.3,22.86 90 bottom
R43  56.64,33.02 90 top
R44  53.34,33.02 270 top
R45  50.04,33.02 270 top
R46  46.35,27.94 270 top
R47  50.04,27.94 90 top
R48  54.23,13.08 270 top
R49  78.11,50.16 180 bottom
R50  78.11,46.99 180 bottom
R51  78.11,43.81 180 bottom
R52  73.03,50.16 180 bottom
R53  73.03,46.99 180 bottom
R54  73.03,43.81 180 bottom
R55  85.09,81.41 90 top
R56  85.09,64.9 90 top
R57  85.09,49.66 90 top
R58  31.11,43.81 270 bottom
R59  27.94,43.81 270 bottom
R60  46.48,62.87 90 top
R61  48.26,47.75 90 bottom
R62  50.8,47.75 270 bottom
R63  43.81,31.24 0 bottom
R64  38.86,31.24 0 bottom
R65  43.81,28.07 0 bottom
R66  38.86,28.07 0 bottom
SW1  43.31,91.31 90 top
SW2  53.34,91.31 90 top
TP1  5.08,93.98 0 top
TP2  5.08,81.28 0 top
TP3  5.08,68.58 0 top
TP4  5.08,55.88 0 top
TP5  5.08,43.18 0 top
TP6  5.08,30.48 0 top
TP7  91.44,76.2 0 top
TP8  91.44,60.96 0 top
TP9  91.44,45.72 0 top
TP10  38.1,101.6 0 top
TP11  58.42,101.6 0 top
TP12  17.78,5.08 0 top
TP13  27.94,5.08 0 top
TP14  91.44,20.32 0 top
TP15  71.12,101.6 0 top
TP16  25.4,101.6 0 top
TP17  5.08,17.78 0 top
TP18  61.09,13.72 0 top
TP19  16,17.78 0 top
TP20  43.94,66.93 0 top
TP21  24.64,89.15 0 top
TP24  27.94,89.28 0 top
TP25  19.68,77.98 0 top
TP26  19.68,65.41 0 top
TP27  19.68,52.58 0 top
TP28  19.68,39.88 0 top
TP29  19.68,27.3 0 top
TP33  40.01,81.28 0 top
TP34  57.15,81.28 0 top
U1  50.8,55.24 0 top
U2  39.88,49.78 0 bottom
U3  30.48,50.16 0 bottom
U4  66.04,47.62 270 bottom
U5  50.8,40.64 270 bottom
U6  67.31,19.68 180 top
U7  29.21,16.51 270 bottom
U8  52.07,20.95 270 top
U$13  [LT_LOGO_LARGE]  67.94,89.28 0 top
U$14  [DC1633_FRAME]  50.8,28.7 0 top
U$20  [DL94570652]  not placed on the board

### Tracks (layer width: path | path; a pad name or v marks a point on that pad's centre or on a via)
+3V3  (via drill 0.25)
  Top 0.178: R60.2 C7.1 50.42,63.72 | 50.42,63.72 50.42,59.31 49.78,58.67 49.78,54.94 48.64,54.94 U1.5 47.18,54.93 46.61,54.36 v46.61,49.53 | 50.42,63.72 R13.2 53.47,63.72 | 53.47,63.72 53.47,61.98 54.86,61.98 R14.2 | 53.47,63.72 v53.47,66.93
  Top 0.203: R60.2 46.48,65.28 44.96,66.93 TP20.1
  Bottom 0.178: v53.47,66.93 59.13,72.09 JP7.1 | v46.61,49.53 46.61,49.28 47.24,48.64 48.22,48.64 R61.2
+5V  (via drill 0.25)
  Top 0.178: 50.8,18.8 50.42,18.8 U8.9 | 53.34,18.8 53.72,18.8 U8.16 53.85,18.67 | 50.8,18.8 50.8,19.43 51.05,19.68 53.09,19.68 53.34,19.43 53.34,18.8 | 50.8,18.8 U8.10 | 53.34,18.8 U8.15 | 61.09,17.53 61.02,16.83 | 82.55,50.55 80.01,50.55 | 82.55,50.55 85.09,50.55 | 82.55,50.55 R29.2 | 85.09,50.55 86.11,50.55 86.61,50.04 v86.61,47.75 | 85.09,50.55 R57.2 | 80.01,65.79 R28.2 R27.2 82.55,65.79 | 82.55,65.79 85.09,65.79 R56.2 | R55.2 85.09,82.3 82.55,82.3 R25.2 81.28,82.26 | 79.88,50.55 80.01,50.55 | 80.01,50.55 R30.2 | R48.2 54.23,13.08 57.28,13.08 57.91,13.72 TP18.TP | v81.28,83.95 81.28,82.26 | R26.2 81.28,82.26 | v81.28,67.06 81.28,65.79 82.55,65.79
  Top 0.254: 79.88,50.55 86.11,50.55 87.25,51.69 87.25,65.02 86.49,65.79 85.13,65.79 R56.2
  Top 0.406: v59.82,18.67 53.85,18.67
  Top 0.61: C24.1 v59.82,18.67 61.09,17.53 TP18.TP
  Route15 0.178: v38.73,60.07 v38.73,58.04
  Bottom 0.178: C15.1 38.73,41.4 v40.64,41.4 43.94,38.1 51.18,38.1 51.69,38.61 51.69,39.24 U5.4 51.82,39.37 55.88,39.37 C20.1 55.88,39.12 58.42,39.12 C17.1 | 78.99,46.99 78.99,43.81 R51.2 | 78.99,50.16 78.99,52.45 69.85,52.45 69.85,49.4 68.2,49.4 U4.1 | 78.99,50.16 78.99,48.64 78.99,46.99 | 78.99,46.99 R50.2 | 78.99,50.16 R49.2 | 34.42,52.2 36.45,51.03 U2.28 | 39.75,57.78 39.75,56.13 37.85,56.13 34.42,52.58 34.42,52.2 | 39.75,60.07 39.75,59.82 40.64,59.82 42.55,61.72 42.55,65.02 40.39,65.02 39.75,65.66 39.75,66.67 R31.2 | 39.75,60.07 39.75,62.23 R32.2 | 39.75,57.78 39.75,58.04 v38.73,58.04 | 39.75,60.07 v38.73,60.07 | 39.75,57.78 R33.2 | C28.1 27.3,52.2 28.83,53.72 31.5,53.72 31.5,52.27 U3.8 31.53,52.2 34.42,52.2
  Bottom 0.203: 79.73,48.64 78.99,48.64 | v58.42,37.34 C17.1
  Bottom 0.254: v86.61,47.75 80.62,47.75 79.73,48.64 | JP1.3 v19.3,95.89
  other vias: 56.64,18.67
  pour Route15: 0.76,0.76 95.25,1.27 95.25,105.41 0.76,105.92
+12V
  Top 0.178: 72.73,18.67 C22.1
  Top 0.254: 71.12,18.67 69.6,18.67 U6.1 | 71.12,18.67 71.12,20.19 70.74,20.57 69.6,20.57 U6.3 | 71.12,18.67 72.73,18.67
  Top 0.305: J2.3 73.66,12.91 C22.1
ADC_CH0  (via drill 0.25)
  Route15 0.178: v44.2,49.66 42.55,51.31 42.55,83.69 36.7,89.28 TP24.1
  Bottom 0.178: v44.2,49.66 43.26,49.66 42.77,49.02 42.29,49.02 42.29,49.03 U2.8 | C1.1 24.77,93.98 24.77,91.44 R7.2 24.64,91.27 24.64,90.17 | R1.1 24.64,90.17 | TP24.1 27.94,90.17 24.64,90.17
ADC_CH1  (via drill 0.25)
  Route15 0.178: v43.43,48.9 41.66,50.67 41.66,81.28 40.39,82.55 39.37,82.55 34.8,77.98 TP25.1
  Bottom 0.178: v43.43,48.9 42.93,48.54 42.29,48.53 U2.9 | R2.1 18.29,78.11 18.92,77.98 TP25.1 21.97,77.98 | 21.97,77.98 21.97,80.64 C2.1 | 21.97,77.98 R8.2
ADC_CH2  (via drill 0.25)
  Top 0.178: v44.2,48.26 42.27,48.26 42.27,48.77 30.58,60.33 v29.97,60.33
  Bottom 0.178: R3.1 TP26.1 21.97,65.41 | v44.2,48.26 43.23,48.26 43.03,48.18 42.8,48.03 U2.10 42.29,48.03 | v29.97,60.33 26.67,63.63 22.73,63.63 21.97,64.39 21.97,65.41 | 21.97,65.41 21.97,67.94 C3.1 | 21.97,65.41 R9.2
ADC_CH3  (via drill 0.25)
  Route2 0.178: v43.31,47.62 39.24,51.31 21.21,51.31 20.57,51.82 TP27.1
  Bottom 0.178: v43.31,47.62 42.29,47.5 42.29,47.53 U2.11 | R4.1 18.29,52.7 18.92,52.58 TP27.1 21.97,52.58 | 21.97,52.58 21.97,55.24 C4.1 | 21.97,52.58 R10.2
ADC_CH4  (via drill 0.25)
  Route2 0.178: v44.07,46.61 36.45,46.61 35.43,45.59 33.78,45.59 27.69,39.88 TP28.1
  Bottom 0.178: v44.07,46.61 42.55,46.61 42.55,46.74 U2.12 | R5.1 18.41,40.01 19.05,39.88 TP28.1 R11.2 C5.1
ADC_CH5
  Bottom 0.178: U2.13 42.93,44.79 42.93,43.43 39.12,43.43 37.97,44.58 34.8,44.58 33.02,42.67 33.02,37.08 31.88,36.07 24.64,28.83 22.01,28.83 | R12.2 22.01,28.83 | 22.01,28.83 C6.1
  Bottom 0.203: R12.2 TP29.1 R6.1
ADC_CH6  (via drill 0.25)
  Top 0.178: 82.55,70.99 v81.28,70.99 80.01,70.99 C12.1 | 82.55,70.99 85.09,70.99 R19.1 | 82.55,70.99 R22.2
  Route2 0.178: v81.28,70.99 77.6,70.99 57.78,51.18 53.98,51.18 47.24,44.45 v41.91,44.45
  Bottom 0.178: U2.14 40.88,45.48 v41.91,44.45
ADC_CH7  (via drill 0.25)
  Top 0.178: 82.55,55.75 80.01,55.75 | v74.8,55.75 80.01,55.75 | 80.01,55.75 C13.1 | 82.55,55.75 85.09,55.75 R20.1 | 82.55,55.75 R23.2
  Route2 0.178: v61.21,59.31 47.12,45.47 41.66,45.47 v40.64,44.45
  Bottom 0.178: v61.21,59.31 71.63,59.31 v74.8,55.75 | U2.15 40.38,44.59 v40.64,44.45
ADC_CH8  (via drill 0.25)
  Top 0.178: 82.55,40.51 80.01,40.51 80.01,40.54 | 82.55,40.51 85.09,40.51 R21.1 | 82.55,40.51 R24.2 | 80.01,40.54 v78.23,40.54 | C14.1 80.01,40.54
  Route2 0.178: v78.23,40.54 75.95,43.43 40.39,43.43 v39.37,44.45
  Bottom 0.178: U2.16 39.88,44.96 v39.37,44.45
ADC_CH9  (via drill 0.25)
  Top 0.178: 37.85,83.44 C10.1 40.01,83.61 | R15.1 R17.2 40.01,83.61 | TP33.1 40.01,83.61
  Route15 0.178: v38.73,45.41 39.12,45.85 39.12,57.53 39.37,57.78 39.37,80.39 TP33.1
  Bottom 0.178: 38.86,45.47 v38.73,45.41 39.38,45.41 U2.17
ADC_CH10  (via drill 0.25)
  Top 0.178: R16.1 R18.2 57.15,83.61 | TP34.1 57.15,83.61 | C11.1 57.15,83.61
  Route2 0.178: v36.83,45.97 37.21,46.23 42.8,46.23 43.05,45.97 44.83,45.97 50.67,51.82 51.31,51.82 56.77,57.28 56.77,80.9 TP34.1
  Bottom 0.178: v36.83,45.97 37.34,45.97 37.88,46.59 38.19,47.02 38.86,47.02 38.88,46.92 U2.18
ADC_CH11  (via drill 0.25)
  Route15 0.178: v37.47,45.21 37.47,44.32 38.23,43.56 43.56,43.56 v46.86,46.86
  Bottom 0.178: R62.2 R61.1 48.22,46.86 v46.86,46.86 | U2.19 37.47,45.42 v37.47,45.21
ADC_CH12  (via drill 0.25)
  Top 0.178: v35.18,46.48 35.18,34.54 v36.83,32.89
  Bottom 0.178: U2.20 35.73,47.03 v35.18,46.48 | v36.83,32.89 39.71,32.89 R64.1 R63.2
ADC_CH13  (via drill 0.25)
  Top 0.178: v34.42,47.12 34.42,31.88 v36.83,29.59
  Bottom 0.178: U2.21 34.83,47.53 v34.42,47.12 | v36.83,29.59 39.71,29.59 R66.1 R65.2
DAC_CH2  (via drill 0.25)
  Route15 0.178: v63.37,55.12 51.56,66.93 v51.56,71.12
  Bottom 0.178: v63.37,55.12 64.14,54.36 65.02,54.36 R39.R2_2 | v51.56,71.12 40.51,82.42 16.38,82.42 JP2.2 JP2.1
DAC_CH3  (via drill 0.25)
  Route15 0.178: v49.91,67.56 v63.88,53.59
  Bottom 0.178: v63.88,53.59 65.02,53.59 R39.R3_2 | v49.91,67.56 47.75,69.72 16.38,69.72 JP3.2
  Bottom 0.203: JP3.2 JP3.1
DAC_CH4  (via drill 0.25)
  Route2 0.178: v50.93,53.21 49.91,54.23 16.64,54.23 JP4.2
  Bottom 0.178: v50.93,53.21 62.99,53.21 63.5,52.7 65.02,52.7 R39.R4_2 | JP4.2 JP4.1
DAC_CH5  (via drill 0.25)
  Route15 0.178: v49.4,44.07 48.39,43.05 18.92,43.05 17.91,44.32 16.26,44.32 JP5.2 JP5.1
  Bottom 0.178: v49.4,44.07 57.4,44.07 62.36,39.12 66.17,39.12 66.93,39.88 R40.R4_1
DAC_CH6  (via drill 0.25)
  Route2 0.178: v59.56,38.23 38.99,38.23 29.97,29.21 14.51,29.21 JP6.1
  Bottom 0.178: v59.56,38.23 68.2,38.23 68.2,40.13 67.44,40.89 67.06,40.89 R40.R3_1
  Bottom 0.203: JP6.1 JP6.2
GND  (via drill 0.25)
  Top 0.178: v38.1,55.12 37.34,55.12 v36.07,56.39 | Q3.4 78.74,45.2 78.74,46.48 77.69,46.48 Q3.1 72.91,46.5 v72.14,45.72 | 47.12,53.98 47.12,52.28 51.78,47.62 v53.34,47.62
  Top 0.203: C23.2 56.64,30.86 54.74,30.86 54.74,33.27 54.23,33.78 53.43,33.78 R44.1
  Top 0.406: U1.6 47.43,54.29 47.12,53.98
  Bottom 0.178: 42.32,51.03 U2.4 43.05,51.03 43.05,50.04 U2.6 U2.7 | 38.48,48.53 38.53,48.53 38.15,48.54 U2.23 U2.22 | v36.07,56.39 36.07,57.44 R36.1 | v72.14,45.72 72.14,46.95 R53.1 | R54.1 72.17,42.46 v72.14,42.42 | R52.1 72.17,51.52 v72.14,51.56
  Bottom 0.203: v38.1,55.12 38.88,53.84 U2.33 | 38.48,48.53 U2.39 40.49,51.03 | U4.16 62.26,49.38 v61.72,49.91 | U7.5 28.7,15.62 28.7,16.26 29.21,16.76 U7.2 | 28.32,46.88 v28.19,46.74
  Bottom 0.254: U2.4 40.49,51.03
  Bottom 0.305: U3.4 28.32,46.88
  other vias: 33.53,52.96 39.88,49.78 44.45,55.75 26.67,66.67 38.1,62.1 55.88,42.55 46.74,38.86 28.19,10.16 25.65,44.45 80.01,74.27 80.01,78.97 56.64,30.25 44.96,60.2
  pour Top: 0.76,105.92 95.76,105.92 95.76,0.76 0.76,0.76
  pour Bottom: 0.76,105.92 95.76,105.92 95.76,0.76 0.76,0.76
  pour Route2: 0.76,0.76 95.76,0.76 95.76,105.92 0.76,105.92
I2C_SCL  (via drill 0.25)
  Top 0.178: 51.56,58.55 51.56,60.58 55.5,60.58 56.26,61.47 56.26,63.25 55.79,63.72 R14.1 | 51.56,58.55 51.56,57.28 52.07,56.77 52.07,55.24 52.4,54.94 53.03,54.94 U1.12 | v50.55,58.55 51.56,58.55 | TP13.TP 35.56,5.08 38.1,7.62 | R38.1 38.1,7.62 | J1.4 51.16,2.17 50.29,3.05 50.29,6.35 49.02,7.62 38.1,7.62
  Route15 0.178: v50.55,58.55 49.4,57.4 49.4,44.96 50.04,44.32 50.04,29.21 28.57,7.75 27.94,7.75 TP13.TP
I2C_SDA  (via drill 0.25)
  Top 0.178: TP12.TP 22.23,5.08 22.21,5.07 25.02,8 32.89,8 35.56,10.67 R37.1 36.36,11.85 36.83,12.32 36.83,14.1 39.75,17.02 39.75,38.61 44.83,43.69 v44.83,52.73 | v51.18,61.09 51.18,61.98 52.07,61.98 R13.1 | v51.18,56.77 51.69,56.26 51.69,55.12 52.45,54.36 53.47,54.36 U1.11
  Bottom 0.178: v51.18,61.09 v51.18,56.77 47.02,52.73 v44.83,52.73 | J1.2 53.26,1.95 52.32,1.02 42.42,1.02 41.02,2.29 20.45,2.29 TP12.TP
N$1  (via drill 0.25)
  Route15 0.178: v62.87,47.5 62.99,47.37 v62.99,41.02
  Bottom 0.178: v62.87,47.5 62.99,47.37 63.88,47.37 U4.12 | v62.99,41.02 64.01,40.01 65.02,40.01 R40.R4_2
N$2
  Bottom 0.178: 73.91,47.37 73.91,46.99 R53.2 | U4.10 64.01,46.35 64.52,46.35 65.91,44.96 72.35,44.96 R53.2 | R50.1 R53.2
N$3  (via drill 0.25)
  Route15 0.178: v65.02,47.62 63.88,46.48 v63.88,41.02
  Bottom 0.178: v65.02,47.62 64.77,47.62 64.52,47.88 64.01,47.88 U4.13 | v63.88,41.02 64.01,40.89 65.02,40.89 R40.R3_2
N$4
  Bottom 0.178: R54.2 R51.1 77.25,44.96 78.11,45.72 78.11,48.26 71.88,48.26 70.48,46.86 70.48,46.35 68.2,46.35 U4.7
N$5  (via drill 0.25)
  Top 0.178: v60.83,47.5 60.45,46.86 v60.45,42.55
  Bottom 0.178: v60.83,47.5 61.47,48.13 63.12,48.13 63.37,48.39 63.88,48.39 U4.14 | v60.45,42.55 61.34,41.66 65.02,41.66 R40.R2_2
N$6
  Bottom 0.178: 73.91,50.16 73.91,49.02 71.88,49.02 69.72,46.86 68.2,46.86 U4.6 | 73.91,50.16 R52.2 | 73.91,50.16 R49.1
N$7  (via drill 0.25)
  Top 0.178: v65.02,44.07 v65.02,46.74
  Bottom 0.178: v65.02,46.74 65.66,46.74 65.66,48.13 65.28,48.51 64.9,48.51 64.52,48.9 64.01,48.9 U4.15 | v65.02,44.07 65.02,42.55 R40.R1_2
N$9  (via drill 0.25)
  Route15 0.178: v67.06,47.37 66.42,48.01 66.42,50.16 v67.18,50.93
  Bottom 0.178: v67.06,47.37 68.07,47.37 U4.5 | v67.18,50.93 67.18,51.69 66.8,52.7 66.93,52.7 R39.R4_1
N$10
  Top 0.178: R48.1 56.01,13.93 LED5.P
N$11  (via drill 0.25)
  Route15 0.178: v69.22,48.39 69.09,48.51 v69.09,50.04
  Bottom 0.178: v69.22,48.39 68.71,47.88 68.2,47.88 U4.4 | v69.09,50.04 68.2,50.93 68.2,53.59 67.06,53.59 R39.R3_1
N$12  (via drill 0.25)
  Top 0.178: U8.2 53.34,23.24 53.72,23.24 U8.1 53.85,23.24 53.85,25.65 54.61,26.42 | C23.1 58.55,26.67 61.85,26.67 | 61.85,26.67 61.98,26.67 | 54.74,26.54 54.61,26.42 | v54.61,27.69 54.61,26.42 | U6.5 63.5,18.73 C34.1 62.57,18.96 61.98,19.56 61.98,26.54 61.85,26.67
  Top 0.203: 54.74,26.54 56.64,26.54 C23.1 | R43.2 57.57,33.87 58.55,32.89 58.55,26.67
  Bottom 0.178: v54.61,27.69 51.05,31.24 R63.1
N$13  (via drill 0.25)
  Route15 0.178: v67.06,48.39 68.2,49.53 v68.2,54.23
  Bottom 0.178: v67.06,48.39 68.07,48.39 U4.3 | v68.2,54.23 68.07,54.36 67.06,54.36 R39.R2_1
N$14
  Top 0.178: R44.2 53.34,32.13 53.21,32.13 53.21,24.26 52.83,23.88 52.83,23.24 U8.3 52.83,23.11 52.83,22.48 52.63,22.23 51.56,22.23 51.31,22.48 51.31,23.11 U8.6
  Top 0.203: R44.2 52.41,32.17 51.82,32.77 51.82,35.69 54.99,35.69 55.5,35.18 | 55.5,35.18 55.5,32.17 R43.1 | C33.1 59.94,34.67 58.93,35.69 56.01,35.69 55.5,35.18
N$15
  Top 0.178: R60.1 45.47,62.02 45.47,63.63 44.58,63.63 LED4.P
N$16
  Bottom 0.178: 31.11,46.86 30.81,46.86 30.81,47.24 U3.2 | 31.11,46.86 31.46,46.86 | R58.1 31.11,46.86 | U3.1 31.46,46.86 | 31.46,46.86 31.47,46.86
N$17
  Bottom 0.203: TP1.TP JP1.1
N$18
  Bottom 0.178: U4.2 68.07,48.9 67.56,48.9 66.17,50.29 66.17,55.24 66.93,55.24 R39.R1_1
N$19  (via drill 0.25)
  Top 0.203: R38.2 38.1,14.22 v43.81,19.94
  Route15 0.178: v51.44,50.93 51.44,27.3 51.18,27.3 v43.81,19.94
  Bottom 0.178: U4.8 68.07,45.85 66.42,45.85 66.42,48.01 63.5,50.93 v51.44,50.93 44.58,50.93 43.41,52.03 U2.2 | U2.2
N$20  (via drill 0.25)
  Top 0.178: 48.51,55.5 U1.4 | JP1.2 17.32,93.95 17.32,92.41 20.57,89.15 TP21.1
  Top 0.203: U1.4 45.4,55.56 44.45,54.61 38.86,54.61 38.86,55.88 38.1,55.88 36.07,57.91 C29.1 v33.87,61.13
  Route2 0.203: v33.87,61.13 20.95,74.04 20.95,87.12 17.3,90.77 JP1.2
  Bottom 0.178: R1.2 18.44,91.31 17.3,92.3 JP1.2
N$21
  Top 0.178: U8.4 52.32,23.24 52.32,28.7 50.04,30.99 R45.2
N$22
  Top 0.178: U8.5 51.82,23.24 51.82,23.88 50.04,26.04 R47.1 R46.2
N$23
  Top 0.178: C34.2 65.69,20.66 U6.4
N$24
  Bottom 0.178: R42.1 27.3,21.97 28.32,21.97 28.32,18.16 U7.1 28.32,18.03 28.32,16.26 28.07,16.26 27.18,15.37 27.18,8.51 38.93,8.51 J1.11
N$25  (via drill 0.25)
  Top 0.178: J1.12 41.77,2.17 41.02,2.92 41.02,4.83 v42.55,6.35
  Bottom 0.178: R41.1 30.48,21.97 30.1,21.97 30.1,18.16 U7.3 30.1,18.03 30.1,16.76 29.97,16.76 29.21,16 29.21,9.14 39.75,9.14 v42.55,6.35
N$26  (via drill 0.25)
  Top 0.203: U1.8 49.28,52.07 v55.24,52.07
  Route2 0.178: v55.24,52.07 66.04,62.99 66.04,68.07 64.77,68.07 JP7.3
  Bottom 0.178: JP7.3 JP7.2
N$27  (via drill 0.25)
  Route15 0.178: v40.39,60.45 v40.39,56.64
  Bottom 0.178: v40.39,56.64 40.87,56.26 U2.37 | v40.39,60.45 41.53,61.59 41.53,62.23 R32.1 41.27,62.23 40.39,63.12 39.75,63.12 39.5,63.37 34.67,63.37 34.67,62.23 R35.2
N$28  (via drill 0.25)
  Route15 0.178: v39.75,55.37 39.75,64.77 v40.64,65.66
  Bottom 0.178: v39.75,55.37 39.75,54.48 40.39,53.98 U2.36 | v40.64,65.66 41.53,66.55 41.53,66.67 | 41.53,66.67 41.53,67.06 40.77,67.82 34.67,67.82 34.67,66.67 R34.2 | 41.53,66.67 R31.1
N$29  (via drill 0.25)
  Top 0.178: R37.2 35.56,14.48 37.21,16.13 v37.97,16.13
  Route15 0.178: v43.81,18.54 57.53,32.13 57.53,42.67 59.82,44.96 59.82,46.23 | 59.82,46.23 v59.82,47.5 | v61.72,46.23 59.82,46.23
  Bottom 0.178: v59.82,47.5 57.02,50.29 44.48,50.32 43.33,51.53 U2.3 | v61.72,46.23 62.1,45.85 63.88,45.85 U4.9 | U2.3 | v37.97,16.13 41.4,16.13 v43.81,18.54
N$30
  Bottom 0.178: U2.38 41.38,54.1 41.53,54.99 41.53,57.78 R33.1 41.27,57.78 40.39,58.67 37.34,58.67 37.08,58.93 34.67,58.93 34.67,57.78 R36.2
N$31  (via drill 0.25)
  Route15 0.178: v32.26,49.28 33.4,48.39 v34.8,48.39
  Bottom 0.178: v34.8,48.39 35.31,48.39 36.7,49.02 36.83,49.02 U2.24 | v32.26,49.28 30.86,49.28 30.1,48.51 30.1,48.13 U3.3
N$32  (via drill 0.25)
  Top 0.178: Q2.5 80.26,61.09 80.52,61.34 80.77,61.34 81.53,60.58 81.53,58.55 | 81.53,58.55 84.84,58.55 84.84,57.66 85.09,57.4 R20.2 | 81.53,58.55 v74.8,58.55 69.6,53.09 69.39,52.88 63.25,52.88 63.04,53.02 U1.9
  Bottom 0.178: TP8.TP 89.15,58.55 v74.8,58.55
N$33
  Bottom 0.178: U2.27 36.83,50.55 30.35,50.55 29.46,51.82 29.46,52.2 U3.5
N$34
  Top 0.178: LED1.4 81.92,76.68 81.61,76.96 Q1.6
N$36  (via drill 0.25)
  Top 0.178: Q2.2 77.72,61.09 77.72,60.45 Q2.3 77.72,60.33 v77.72,59.69 | LED2.2 82.93,60.83 82.8,60.71 82.8,60.07 v82.68,59.94 82.68,59.56 85.47,59.56 86.11,60.2 86.11,61.98 85.22,62.87 85.22,64.01 85.09,64.01 R56.1
  Bottom 0.178: v77.72,59.69 82.42,59.69 v82.68,59.94
N$37  (via drill 0.25)
  Top 0.178: Q3.3 77.72,45.21 77.72,45.85 Q3.2 | v82.8,44.45 82.8,45.47 82.93,45.59 LED3.2 83.06,45.47 83.57,45.47 84.07,44.96 85.22,44.96 86.11,45.85 86.11,46.74 85.22,47.62 85.22,48.77 85.09,48.77 R57.1 | 77.72,45.09 Q3.3 | v80.52,44.45 77.98,44.45 77.72,44.7 77.72,45.16 Q3.3
  Bottom 0.178: v82.8,44.45 v80.52,44.45
N$38  (via drill 0.25)
  Top 0.178: v84.96,79.5 84.96,80.52 85.09,80.52 R55.1 | Q1.3 77.72,75.69 77.7,75.69
  Top 0.203: Q1.2 77.7,75.69 v77.72,74.93 | v82.93,74.93 LED1.2
  Bottom 0.178: v77.72,74.93 v82.93,74.93 84.96,76.96 v84.96,79.5
N$39
  Bottom 0.178: R59.1 27.94,45.72 27.43,46.23 27.43,47.5 28.57,48.64 28.57,52.7 29.21,53.34 30.16,53.34 | 30.16,53.34 U3.6 | U3.7 30.86,52.27 30.86,53.34 30.16,53.34
N$40  (via drill 0.25)
  Top 0.178: Q3.5 80.77,45.85 81.28,45.34 81.28,44.96 82.42,43.81 84.07,43.81 84.07,43.56 84.84,42.8 84.84,42.42 85.09,42.16 R21.2 85.09,42.29 86.11,42.29 88.9,45.59 91.44,45.59 TP9.TP | U1.7 49.59,53.66 v50.04,53.21
  Bottom 0.178: v50.04,53.21 50.8,53.98 61.09,53.98 63.5,56.52 72.26,56.52 74.3,54.48 84.96,54.48 91.44,48.64 TP9.TP
N$41
  Top 0.178: Q1.5 81.41,76.33 81.41,74.04 85.09,74.04 | 85.09,74.04 R19.2 86.96,72.73 87,72.77 87,68.45 86.87,68.33 74.04,68.33 59.37,53.66 U1.10 | TP7.TP 87.12,76.2 85.09,74.04
N$43  (via drill 0.25)
  Top 0.178: v48.39,28.83 49.53,28.83 R47.2
  Bottom 0.178: 30.48,23.75 27.3,23.75 R42.2 | v48.39,28.83 43.31,23.75 31.62,23.75 | 30.48,23.75 31.62,23.75 | 30.48,23.75 R41.2 | 31.62,23.75 31.62,17.14 30.86,16.38 30.1,16.38 30.1,15.24 U7.4 30.1,15.11 30.1,12.06 C26.1 30.06,9.95 30.1,9.91 40.26,9.91 44.2,5.97 47.47,5.97 J1.5
N$44
  Top 0.178: Q3.6 79.88,46.48 81.53,46.48 82.04,46.23 82.68,46.23 82.68,46.1 82.8,46.23 82.93,46.23 LED3.4
N$45
  Top 0.178: LED3.1 84.71,45.47 85.09,45.47 85.47,45.85 85.47,46.48 84.58,47.37 83.44,47.37 82.68,48.13 82.68,48.77 82.55,48.9 R29.1
N$46
  Bottom 0.178: U2.26 34.92,50.03 33.15,48.39 33.15,44.45 32.51,43.81 29.97,43.81 29.21,43.05 28.03,43.05 R59.2 C27.1
N$47
  Top 0.178: LED3.3 84.58,46.23 84.07,46.23 82.93,47.37 80.77,47.37 80.01,48.01 R30.1 80.01,48.9
N$48
  Bottom 0.178: C19.1 R58.2 32.42,42.97 33.66,44.2 33.66,48.26 35.05,49.53 U2.25
N$49
  Top 0.178: Q2.6 79.88,61.72 81.53,61.72 82.04,61.21 82.68,61.21 82.68,61.34 82.8,61.47 82.93,61.47 LED2.4
N$50
  Top 0.178: LED2.1 84.71,60.71 85.09,60.71 85.47,61.09 85.47,61.72 84.58,62.61 83.44,62.61 82.68,63.37 82.68,64.01 82.55,64.14 R27.1
N$51
  Top 0.178: LED2.3 84.58,61.47 84.07,61.47 82.93,62.61 80.77,62.61 80.01,63.37 R28.1 80.01,64.14
N$54
  Top 0.178: LED1.1 84.71,75.95 85.09,75.95 85.47,76.33 85.47,76.96 85.22,77.22 84.84,77.22 82.68,79.38 82.68,80.52 82.55,80.64 R25.1
N$55
  Top 0.178: LED1.3 84.58,76.71 84.07,76.71 80.26,80.52 80.01,80.52 R26.1
N$77
  Top 0.178: 45.59,85.34 45.72,85.34 | 44.96,85.34 45.59,85.34 | 45.59,85.34 R15.2 | 45.72,85.34 46.1,85.34 57.4,76.83 57.4,61.21 56.26,59.82 56.26,56.21 U1.14 | 45.72,85.34 R15.2 | TP10.TP 38.1,92.08 41.1,89.08 41.1,88.3 | C8.1 41.1,88.3 | R15.2 43.31,86.45 SW1.SW1 43.3,88.3 41.1,88.3
N$78
  Top 0.178: U1.13 53.09,55.58 56.64,55.58 56.64,57.91 58.29,59.56 58.29,79.25 61.34,82.55 61.34,85.89 C9.1 55.37,88.3 | TP11.TP 58.42,92.08 58.29,92.08 55.37,89.15 55.37,88.3 | R16.2 53.34,86.58 SW2.SW1 53.42,89.15 53.42,88.3 55.37,88.3
USB_5V  (via drill 0.25)
  Top 0.178: U8.7 50.8,23.24 50.42,23.24 U8.8 50.29,23.24 49.91,23.24 v49.28,22.48 46.39,22.48 C25.1
  Bottom 0.178: J1.1 49.28,8.16 v49.28,22.48 49.28,29.21 48.77,29.72 45.34,29.72 44.66,29.04 R65.1
VIN2
  Top 0.178: U1.3 48.13,56.26 45.47,56.26 41.78,58.42 41.78,62.23 24.64,79.38 19.05,79.38 17.27,81.28 JP2.3
  Bottom 0.178: 15.62,80.01 15.62,78.11 R2.2 15.67,78.02 15.67,76.66 C30.1 | TP2.TP 8.89,81.28 10.16,80.01 15.62,80.01 | 15.62,80.01 15.97,80.01 JP2.3
VIN3  (via drill 0.25)
  Top 0.178: v46.86,59.18 46.86,57.4 47.37,56.9 48.13,56.9 U1.2
  Bottom 0.178: TP3.TP 8.89,68.58 10.29,67.31 15.62,67.31 | 15.62,67.31 15.62,65.41 | 15.62,67.31 16,67.31 16,67.34 JP3.3 | v46.86,59.18 43.43,59.18 43.05,59.44 37.59,59.44 37.34,59.69 29.46,59.69 26.04,62.99 23.75,62.99 | 15.62,65.41 15.62,64.16 16.89,62.99 23.75,62.99 | 15.62,65.41 R3.2 | C31.1 23.75,62.99
VIN4  (via drill 0.25)
  Top 0.178: v47.75,58.29 47.75,57.53 48.13,57.53 U1.1
  Bottom 0.178: 15.62,54.61 15.62,52.7 R4.2 | v47.75,58.29 47.24,58.42 42.93,58.42 42.29,59.05 37.47,59.05 37.21,59.31 28.96,59.31 | 28.96,59.31 23.62,59.31 18.29,54.61 17.27,54.61 | 15.62,54.61 17.27,54.61 | TP4.TP 8.89,55.88 10.16,54.61 15.62,54.61 | 17.24,54.64 17.27,54.61 | JP4.3 17.27,55.88 17.27,54.61 | C32.1 28.96,59.31
VIN5  (via drill 0.25)  (1 unrouted)
  Top 0.178: U1.16 v53.47,59.69
  Route2 0.178: v53.47,59.69 51.18,57.4 v38.1,57.4
  Bottom 0.178: 15.62,41.91 15.62,40.01 R5.2 | v38.1,57.4 35.05,54.36 28.29,54.36 JP5.3 | 15.62,41.91 10.16,41.91 8.89,43.18 TP5.TP | JP5.3 17.25,41.91 15.62,41.91
VIN6  (via drill 0.25)  (1 unrouted)
  Top 0.178: U1.15 54.48,56.83 v54.74,57.53
  Route2 0.178: JP6.3 17.25,38.89 26.16,47.75 41.4,47.75 42.14,47.02 43.54,47.02 43.99,47.37 45.01,47.37 45.01,49.53 47.93,52.45 51.05,52.45 51.82,53.21 51.82,54.61 v54.74,57.53
  Bottom 0.178: 15.62,29.21 15.62,27.3 R6.2 | TP6.TP 8.94,30.48 10.21,29.21 15.62,29.21 | JP6.3 15.97,29.21 15.62,29.21
VREF  (via drill 0.25)
  Top 0.178: v36.07,43.81 v36.07,51.94
  Bottom 0.178: v36.07,51.94 36.65,51.54 U2.29 | 48.64,40.89 49.91,39.62 49.91,39.37 U5.6 | 48.64,40.89 46.23,40.89 45.59,41.48 44.49,41.48 C21.1 44.45,41.78 43.56,42.67 39.12,42.67 37.97,43.81 v36.07,43.81 34.92,43.81 C16.1 35.85,41.49 36.58,40.77 36.58,38.35 TP19.TP1 | U4.11 56.16,46.88 C18.1 56.13,44.96 49.28,44.96 48.64,44.32 48.64,40.89
(copper drawn outside any net)
  shapes: Top area x2

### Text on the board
tSilk: GND | GND | GPI1 | GPI2 | 6V MAX | 6V MAX | (408) 432-1900 | V1 / TEST / POINT | V1 | EXT | EXT | 5V | 14V MAX | V1 | INT | www.linear.com | V2 | EXT | INT | POWERING / THE LTC2933 | 6V MAX | ASEL | V1 | 3.4V-13.9V | V2 | 3.4V-5.8V | H | GPIO1 | 14V MAX | V3 | 3.4V-5.8V | +3.3V / OUT | Z | V4 | 3.4V-5.8V | L | V3 | EXT | INT | 6V MAX | PIN | 1 | GPIO2 | 14V MAX | INT | V4 | EXT | 6V MAX | LTC2933 | PROGRAMMABLE HEX VOLTAGE / SUPERVISOR WITH EEPROM | GPIO3 | V5 | EXT | INT | DEMO CIRCUIT 1633B | 14V MAX | 6V MAX | GPIO LEDs | BLUE=HIGH / RED=LOW | V6 | EXT | INT | 6V MAX | GND | VREF | GND | +5V | 6-14V | SDA | SCL | - | +
bSilk: LTC CONFIDENTIAL FOR CUSTOMER USE ONLY | DATA ACQUISTION SECTION / FOR DEMO EVALUATION | REV 1
d_FabDrawing: 4.20" | 0.00" | 0.00" | 3.80"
